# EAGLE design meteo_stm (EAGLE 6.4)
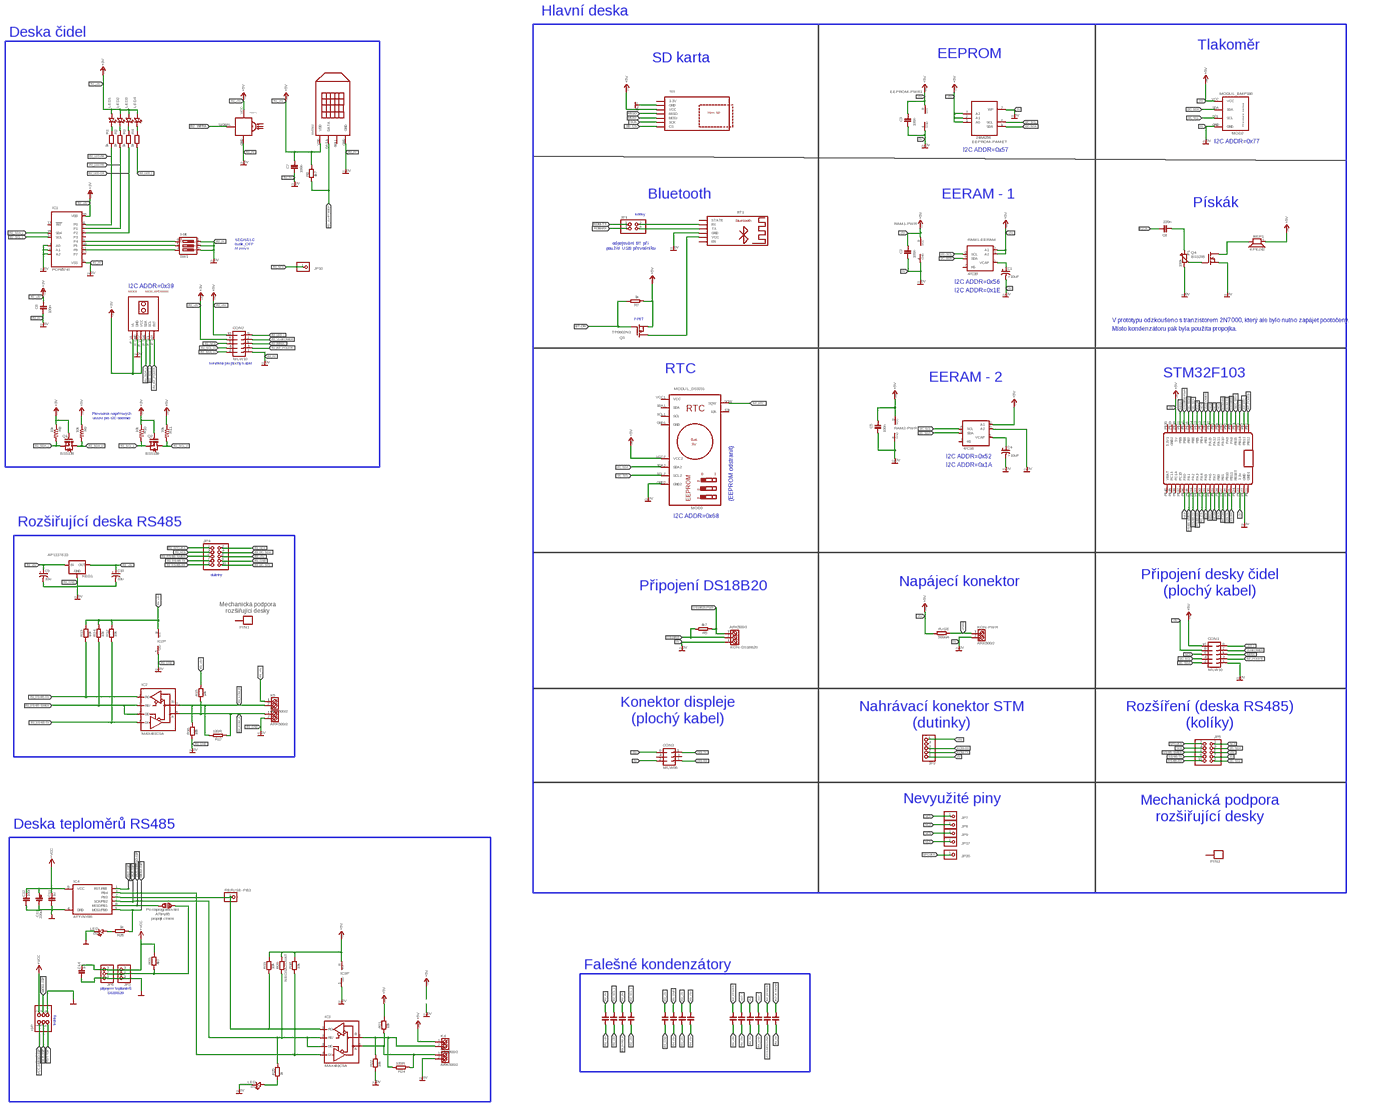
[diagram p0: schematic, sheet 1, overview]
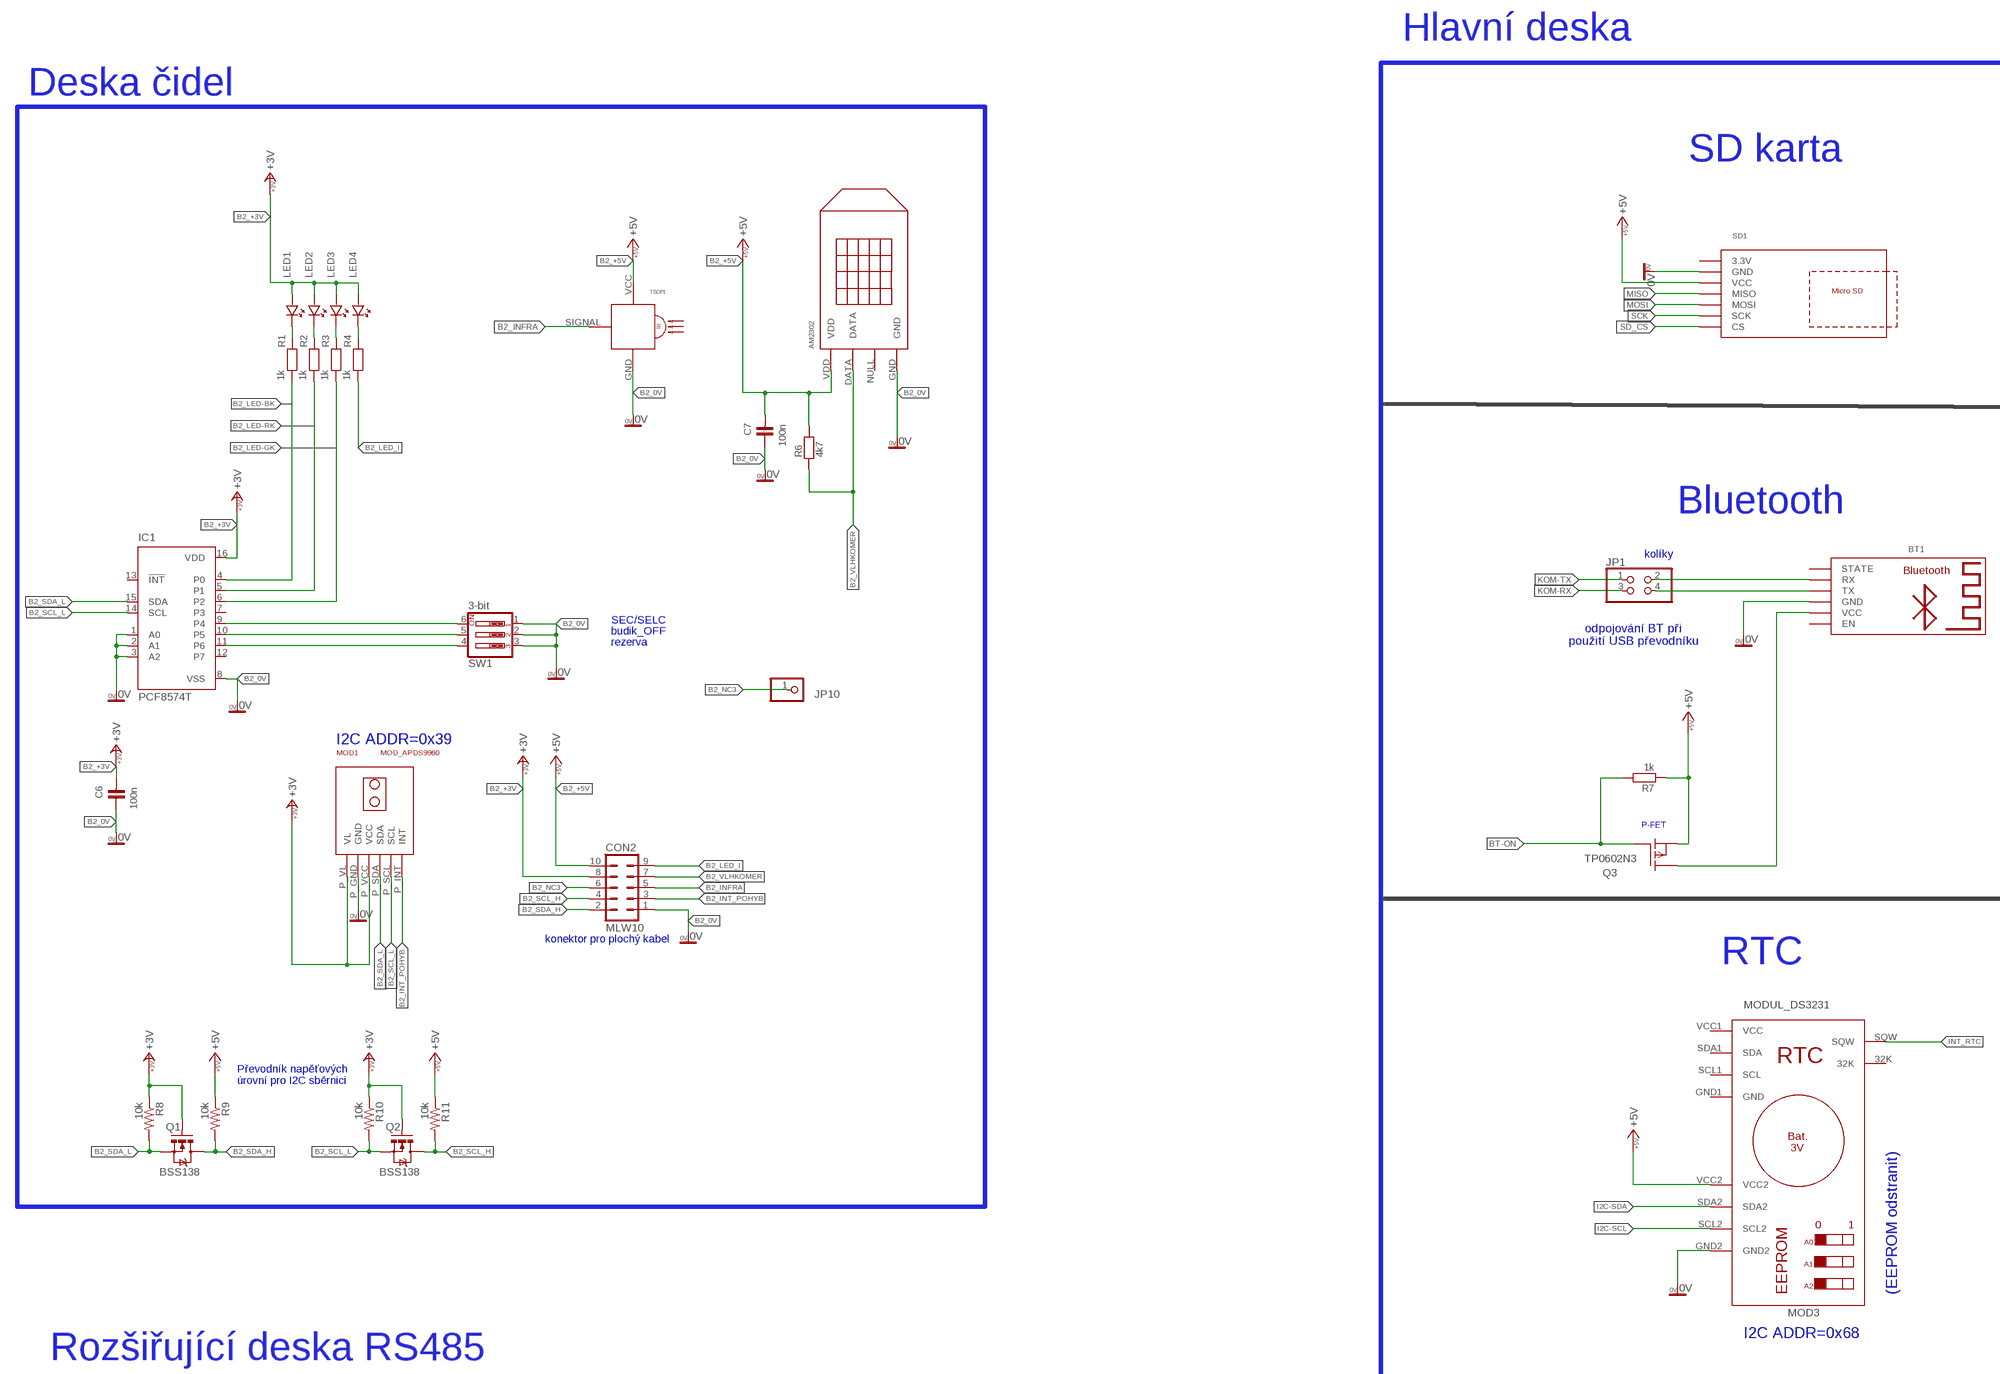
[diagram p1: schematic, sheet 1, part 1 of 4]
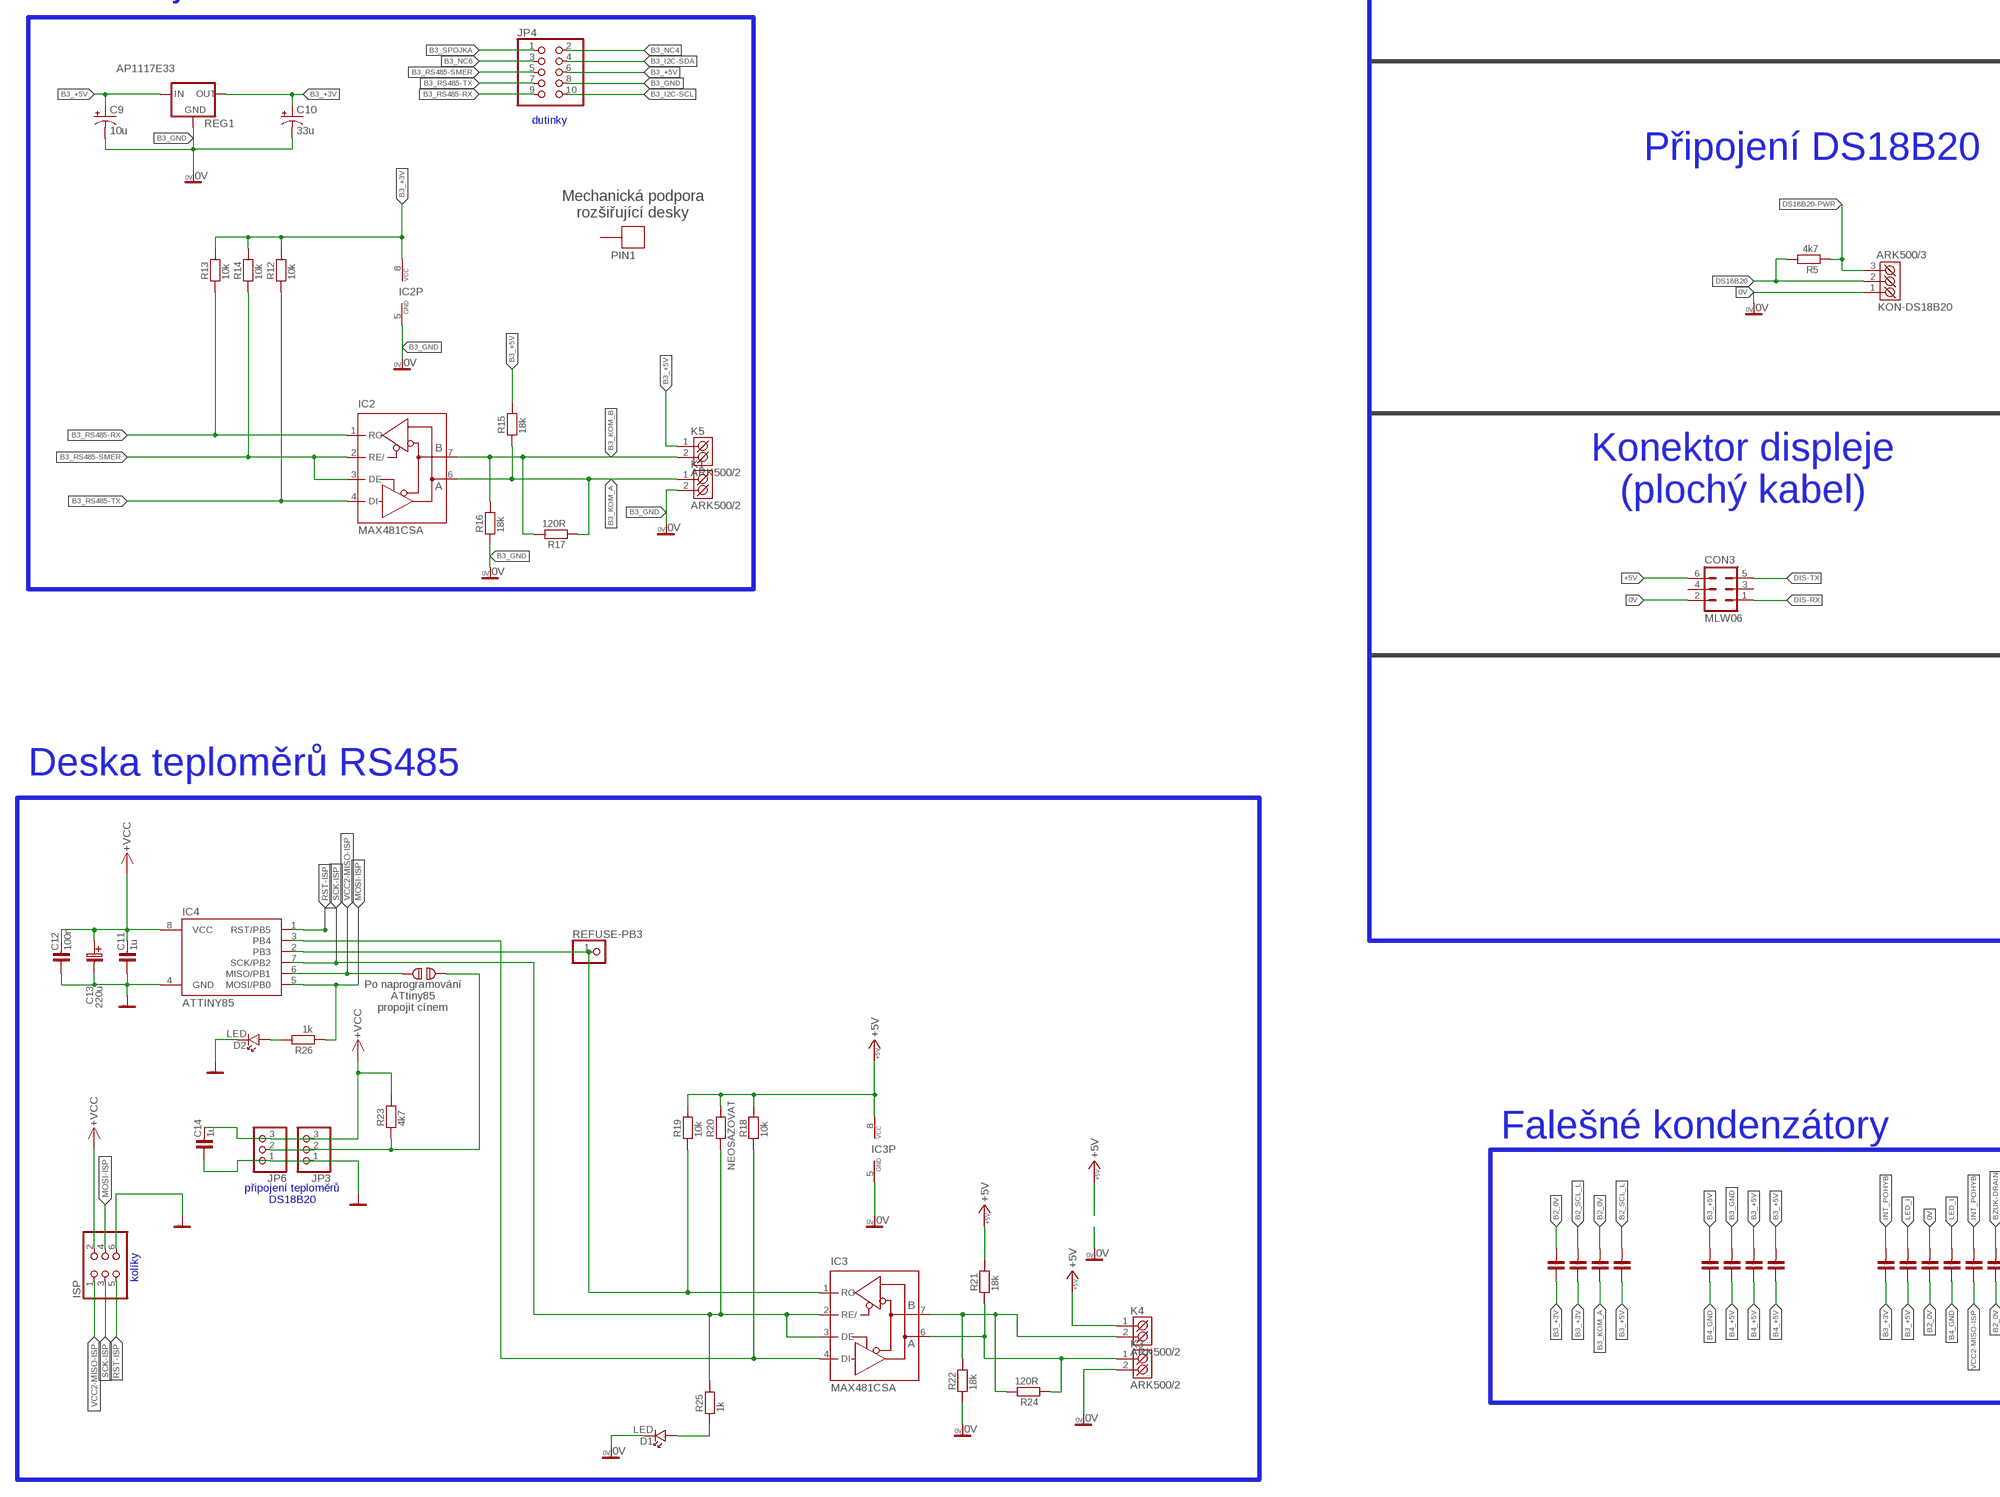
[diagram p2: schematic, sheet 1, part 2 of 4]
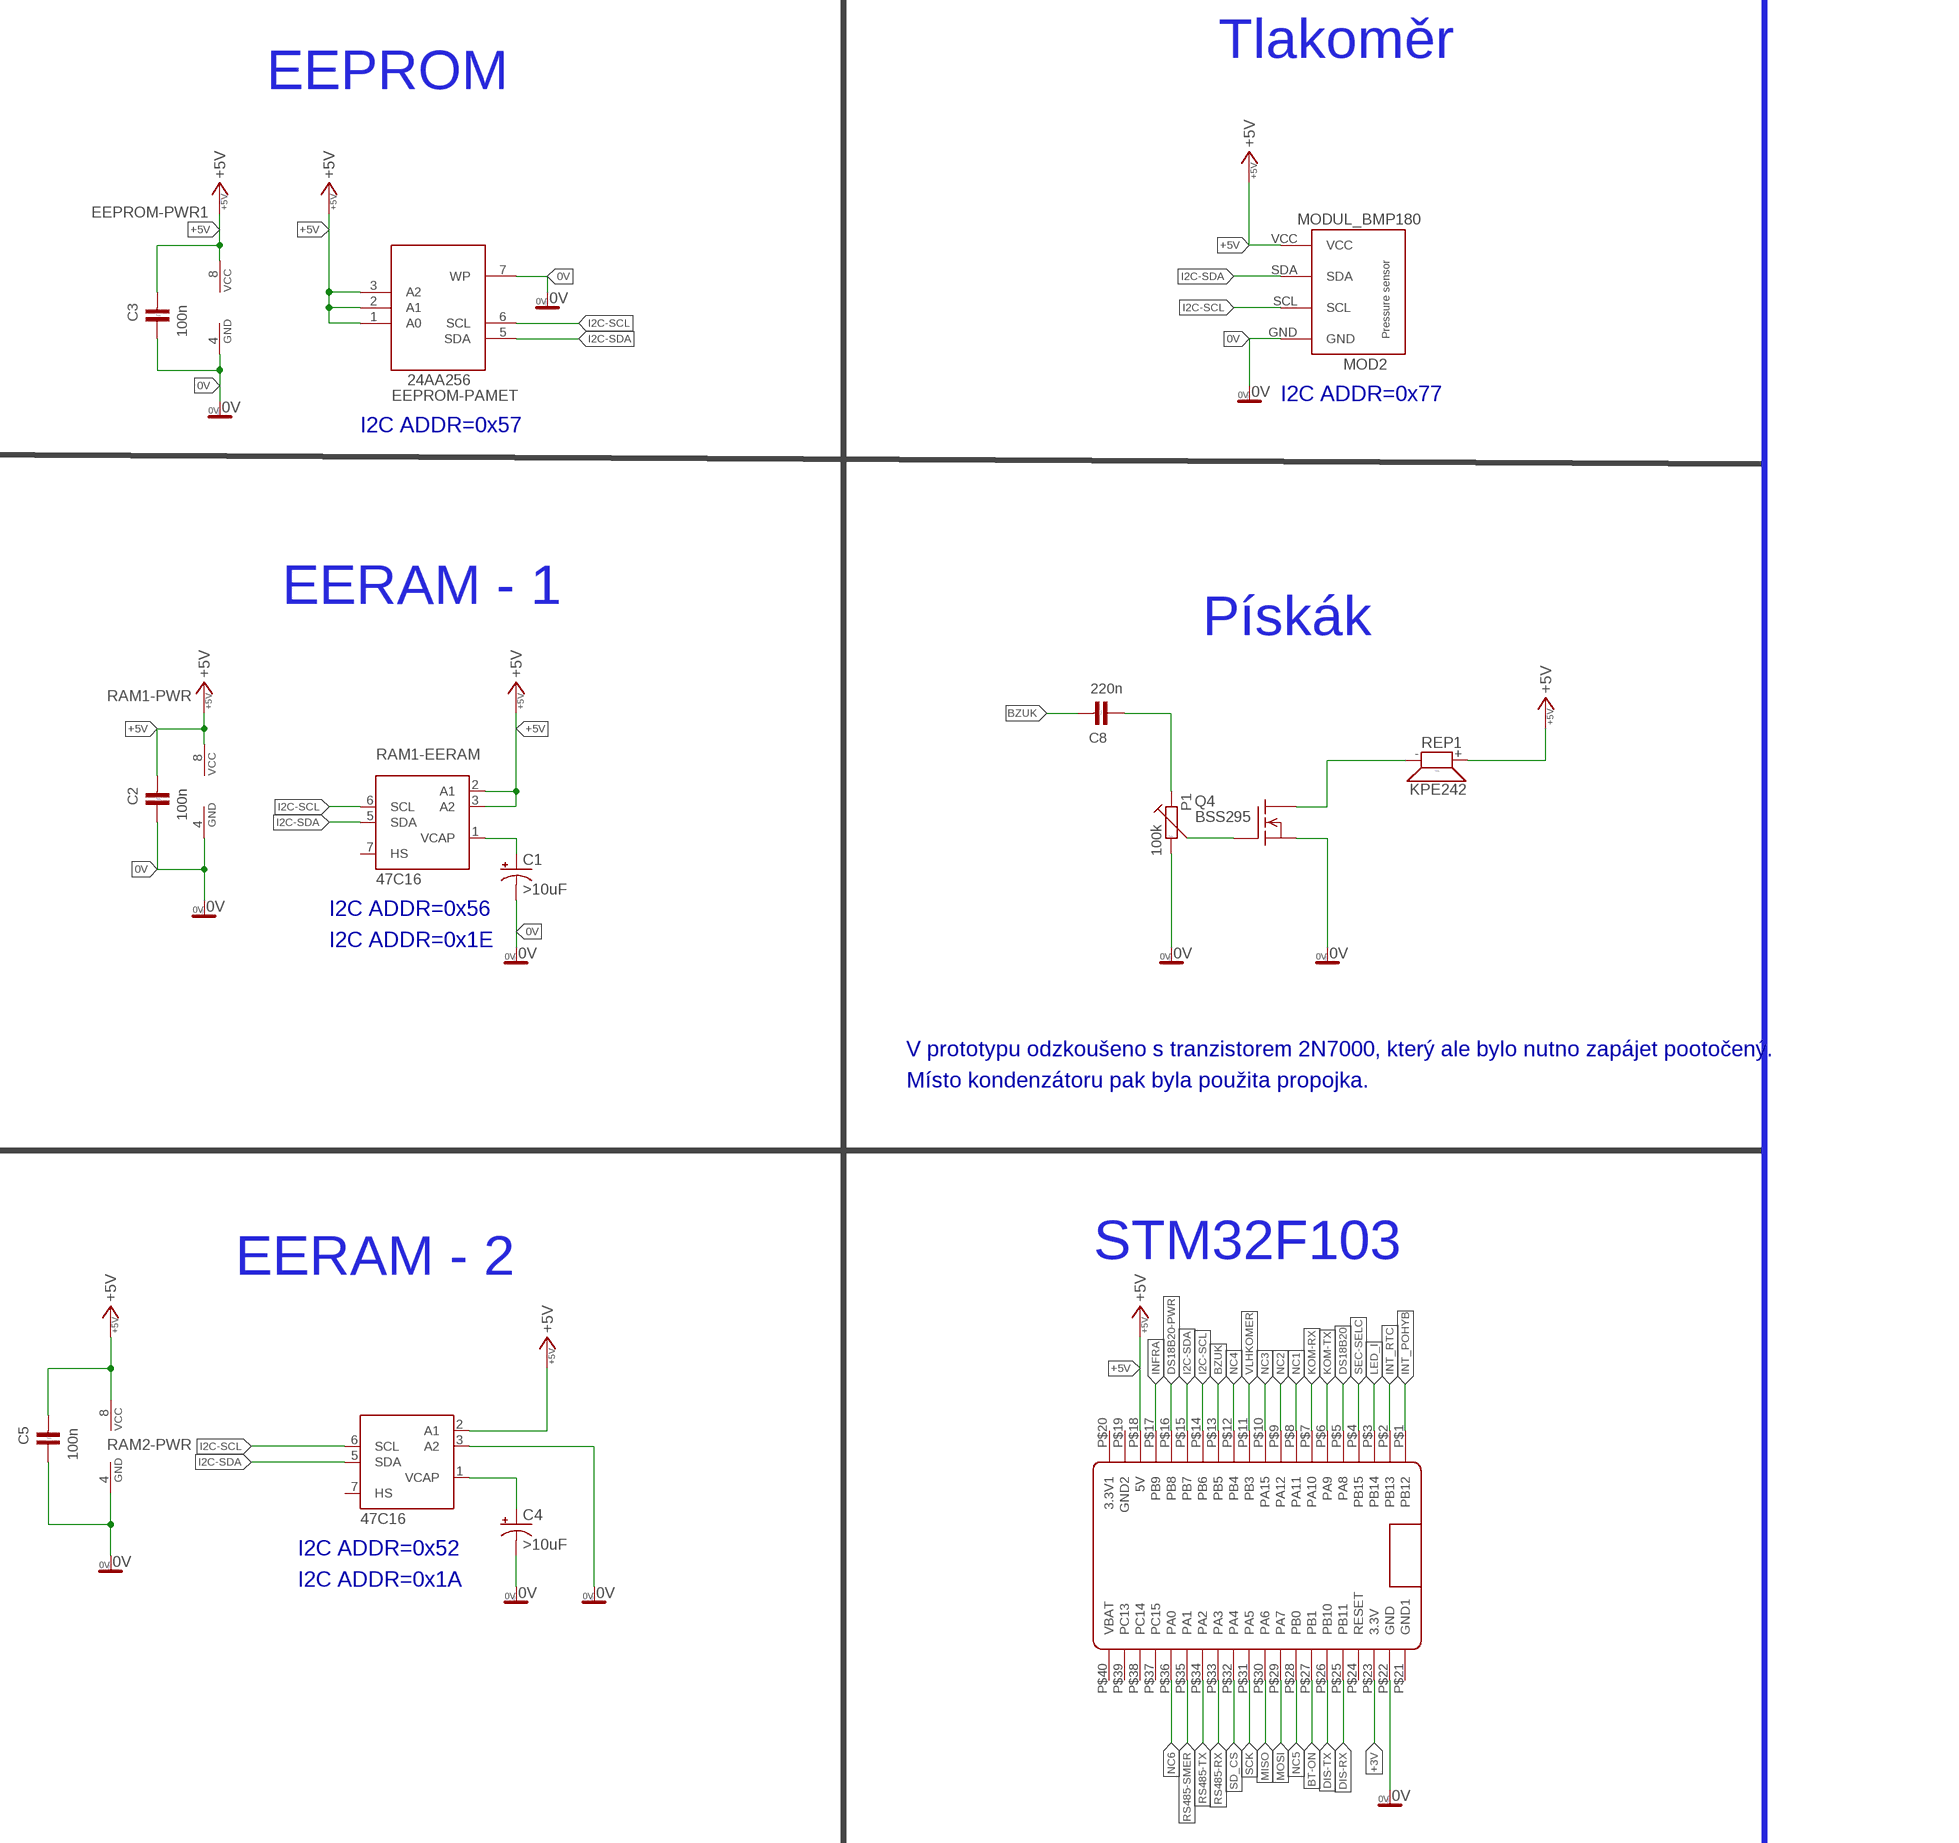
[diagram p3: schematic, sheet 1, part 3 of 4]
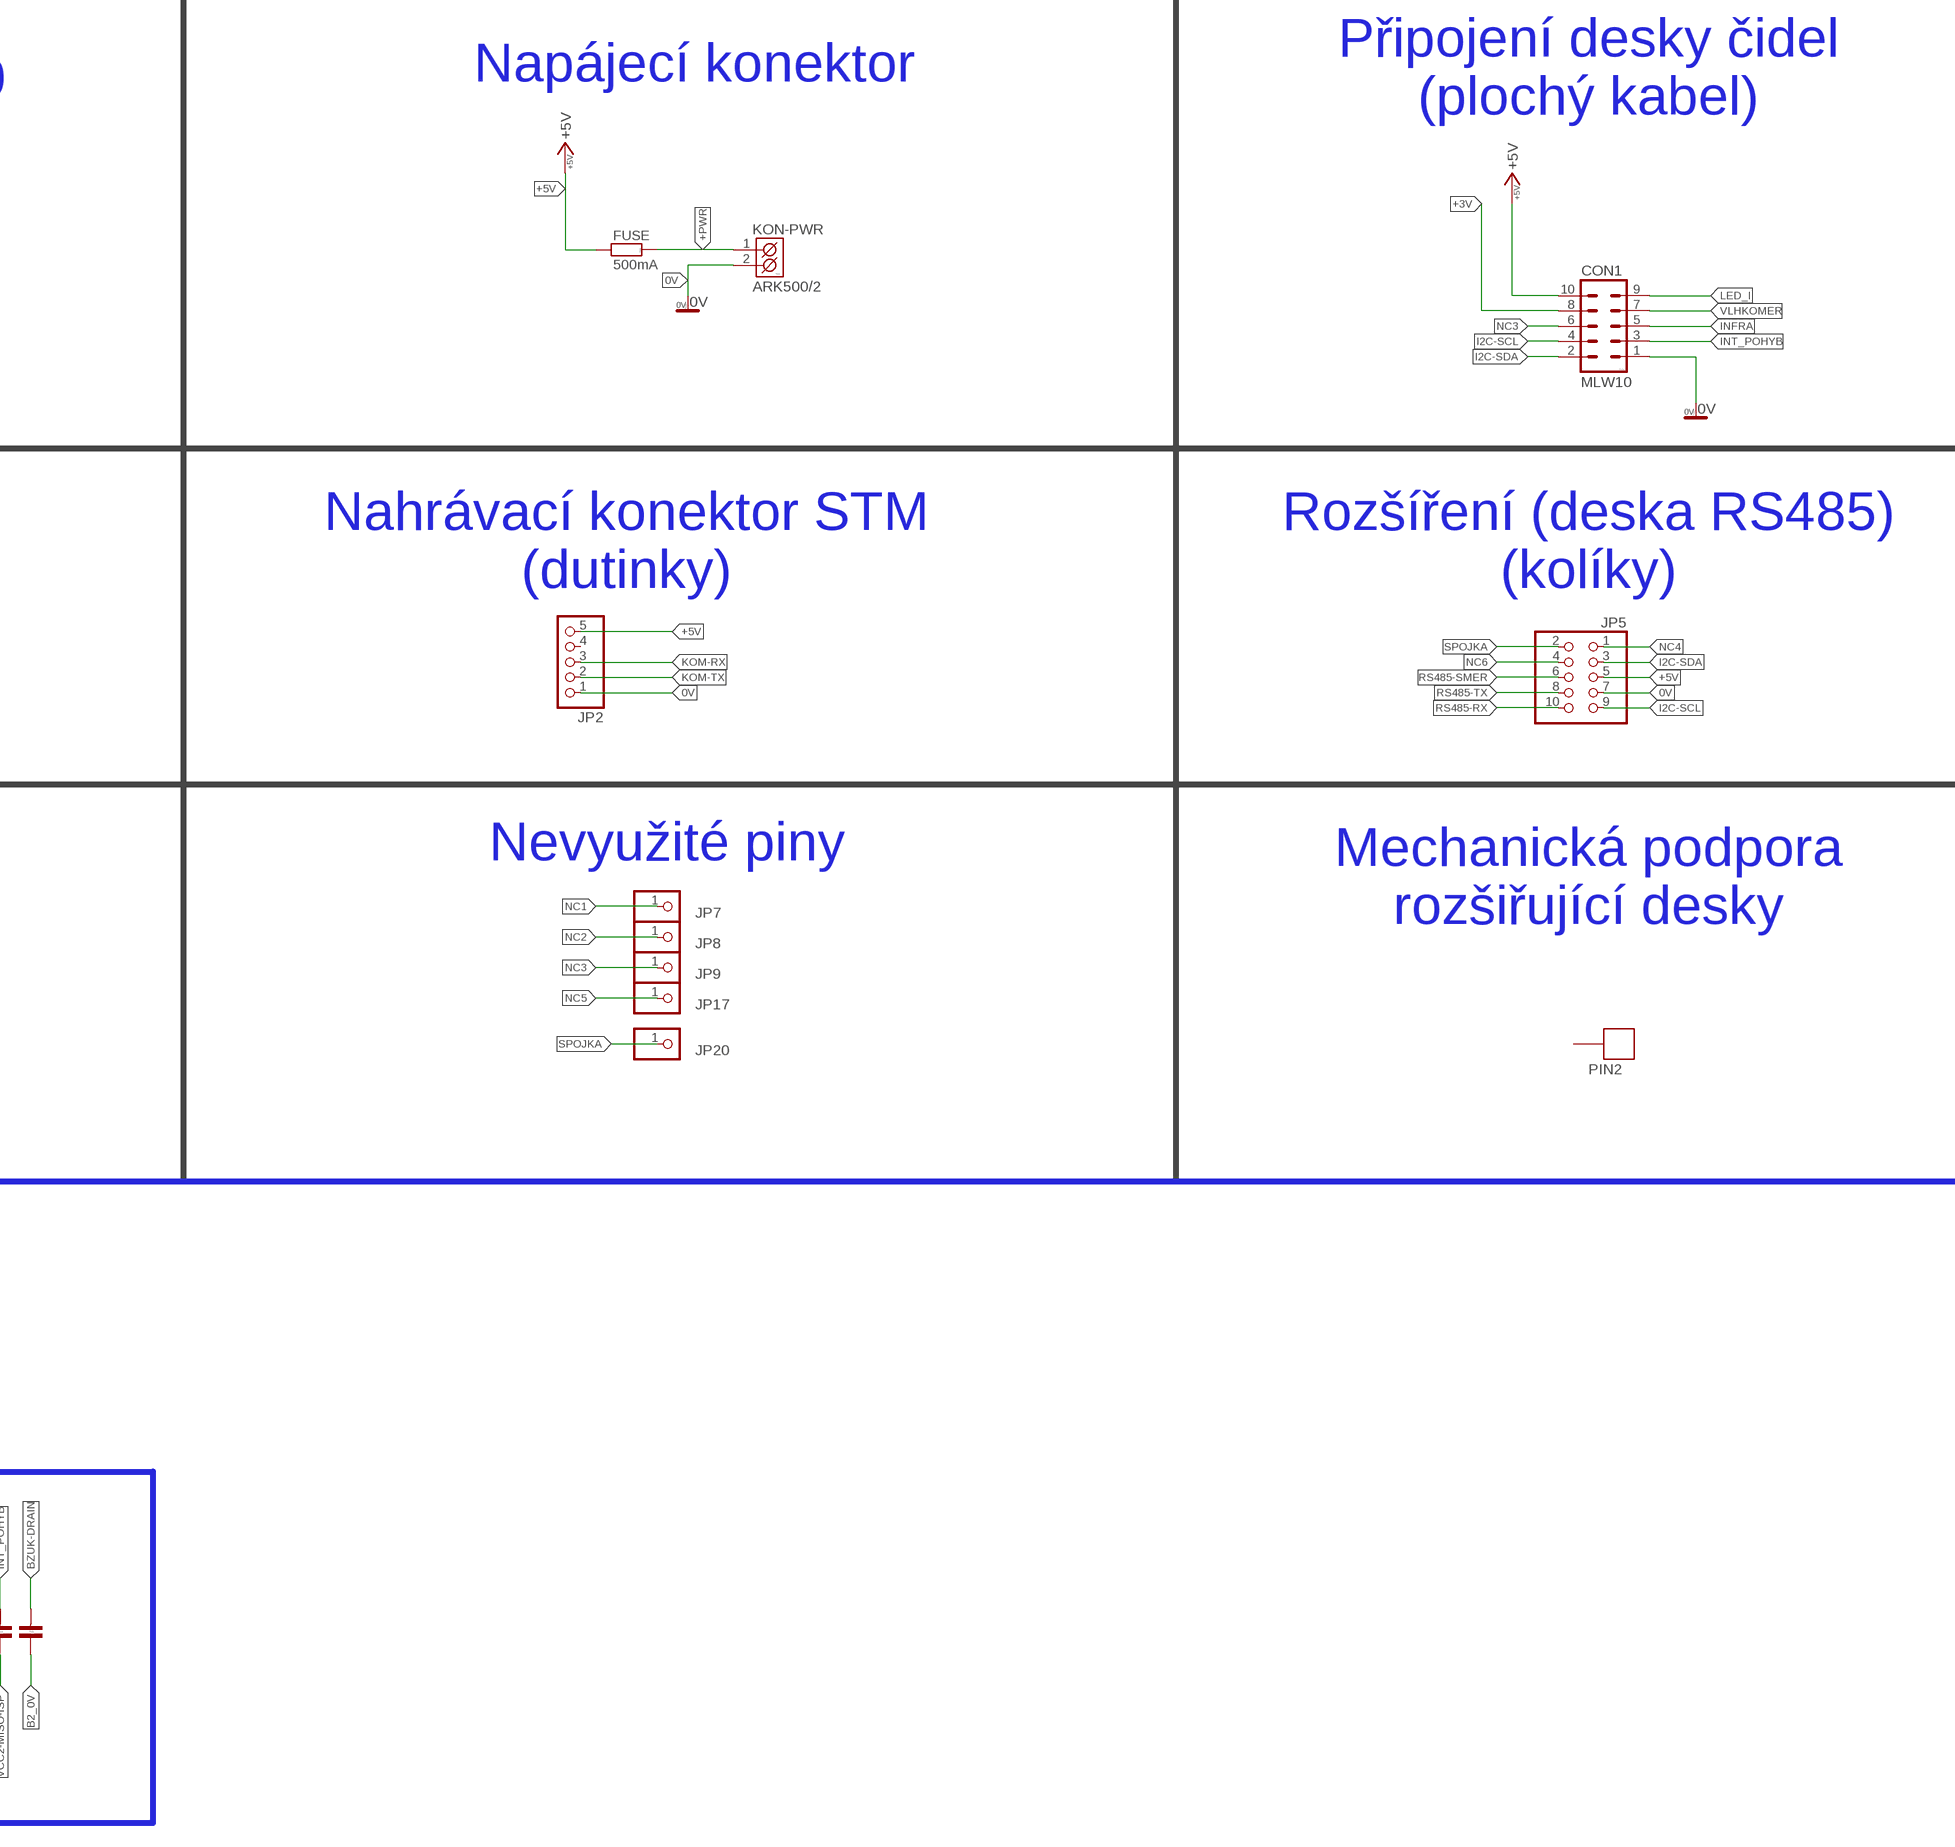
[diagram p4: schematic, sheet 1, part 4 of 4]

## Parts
AM2302  RHT03_DHT-22_AM2302RA  [RHT03_DHT-22/RA]
BT1  BT_MODUL  [BT_MODUL]
C1  >10uF  10UF-POLAR-RADIAL-2.5MM-25V-20%  [CPOL-RADIAL-2.5MM-5MM]
C2  100n  C-KERAMIK_SMD_0805  [0805]
C3  100n  C-KERAMIK_SMD_0805  [0805]
C4  >10uF  10UF-POLAR-RADIAL-2.5MM-25V-20%  [CPOL-RADIAL-2.5MM-5MM]
C5  100n  C-KERAMIK_SMD_0805  [0805]
C6  100n  C-KERAMIK_SMD_0805  [0805]
C7  100n  C-KERAMIK_SMD_0805  [0805]
C8  220n  C-KERAMIK_SMD_0805  [0805]
C9  10u  10UF-POLAR-RADIAL-2.5MM-25V-20%  [CPOL-RADIAL-2.5MM-5MM]
C10  33u  10UF-POLAR-RADIAL-2.5MM-25V-20%  [CPOL-RADIAL-2.5MM-5MM]
C11  1u  C-KERAMIK_SMD_0805  [0805]
C12  100n  C-KERAMIK_SMD_0805  [0805]
C13  220u  C-ELEKTROLYT_3,5  [C-EL_3,5]
C14  1u  C-KERAMIK_SMD_0805  [0805]
C15  ---  C-KERAMIK_SMD_0805  [0805]
C16  ---  C-KERAMIK_SMD_0805  [0805]
C17  ---  C-KERAMIK_SMD_0805  [0805]
C18  ---  C-KERAMIK_SMD_0805  [0805]
C19  ---  C-KERAMIK_SMD_0805  [0805]
C20  ---  C-KERAMIK_SMD_0805  [0805]
C21  ---  C-KERAMIK_SMD_0805  [0805]
C22  ---  C-KERAMIK_SMD_0805  [0805]
C23  ---  C-KERAMIK_SMD_0805  [0805]
C24  ---  C-KERAMIK_SMD_0805  [0805]
C25  ---  C-KERAMIK_SMD_0805  [0805]
C26  ---  C-KERAMIK_SMD_0805  [0805]
C27  ---  C-KERAMIK_SMD_0805  [0805]
C28  ---  C-KERAMIK_SMD_0805  [0805]
CON1  MLW10  [MLW10G]
CON2  MLW10  [MLW10G]
CON3  MLW06  [MLW06G]
D1  LED  LED_SMD_1206  [P1206]
D2  LED  LED_SMD_1206  [P1206]
EEPROM  24AA256  EEPROM  [SO8]
FUSE  500mA  R_SMD_1206  [1206]
IC1  PCF8574T  [SO16W]
IC2  MAX481CSA  [SO08]
IC3  MAX481CSA  [SO08]
IC4  ATTINY85  ATTINY85SU  [ATTINY85]
ISP  PINHD-2X3  [2X03]
JP1  PINHD-2X2  [2X02]
JP2  PINHD-1X5  [1X05]
JP3  PINHD-1X3  [1X03]
JP4  PINHD-2X5  [2X05]
JP5  PINHD-2X5  [2X05]
JP6  PINHD-1X3  [1X03]
JP7  PINHD-1X1  [1X01]
JP8  PINHD-1X1  [1X01]
JP9  PINHD-1X1  [1X01]
JP10  PINHD-1X1  [1X01]
JP17  PINHD-1X1  [1X01]
JP20  PINHD-1X1  [1X01]
K1  ARK500/2  [ARK500/2]
K3  ARK500/2  [ARK500/2]
K4  ARK500/2  [ARK500/2]
K5  ARK500/2  [ARK500/2]
KON-DS18B20  ARK500/3  [ARK500/3]
KON-PWR  ARK500/2  [ARK500/2]
LED1  Modra  LED_3  [LED_3]
LED2  Cervena  LED_3  [LED_3]
LED3  Zelena  LED_3  [LED_3]
LED4  Bila  LED_3  [LED_3]
MOD1  MOD_APDS9960  [MOD_APDS9960]
MOD2  MODUL_BMP180  [MODUL_BMP180]
MOD3  MODUL_DS3231  [DS3231]
P1  100k  TRIMR64Y  [64Y]
PIN1  BIGPIN  [BIGPIN]
PIN2  BIGPIN  [BIGPIN]
Q1  BSS138  MOSFET-NCHANNELSMD  [SOT23-3]
Q2  BSS138  MOSFET-NCHANNELSMD  [SOT23-3]
Q3  TP0602N3  [TO-92]
Q4  BSS295  [TO92]
R1  1k  R_SMD_0805  [0805]
R2  1k  R_SMD_0805  [0805]
R3  1k  R_SMD_0805  [0805]
R4  1k  R_SMD_0805  [0805]
R5  4k7  R_SMD_0805  [0805]
R6  4k7  R_SMD_0805  [0805]
R7  1k  R_SMD_0805  [0805]
R8  10k  RESISTOR0805-RES  [0805]
R9  10k  RESISTOR0805-RES  [0805]
R10  10k  RESISTOR0805-RES  [0805]
R11  10k  RESISTOR0805-RES  [0805]
R12  10k  R_SMD_0805  [0805]
R13  10k  R_SMD_0805  [0805]
R14  10k  R_SMD_0805  [0805]
R15  18k  R_SMD_0805  [0805]
R16  18k  R_SMD_0805  [0805]
R17  120R  R_SMD_0805  [0805]
R18  10k  R_SMD_0805  [0805]
R19  10k  R_SMD_0805  [0805]
R20  NEOSAZOVAT  R_SMD_0805  [0805]
R21  18k  R_SMD_0805  [0805]
R22  18k  R_SMD_0805  [0805]
R23  4k7  R_SMD_0805  [0805]
R24  120R  R_SMD_0805  [0805]
R25  1k  R_SMD_0805  [0805]
R26  1k  R_SMD_0805  [0805]
RAM1  47C16  PCA8581CT  [SO08]
RAM2  47C16  PCA8581CT  [SO08]
REFUSE-PB3  PINHD-1X1  [1X01]
REG1  AP1117E33  V_REG_LD1117VXXLD1117-SMD  [SOT223]
REP1  KPE242  [KPE242]
SD1  MICROSD_MODUL  [MICROSD_MODUL]
SJ-SCL1  SJ  SOLDERJUMPER  [SJ_2S-NO]
SW1  3-bit  SW_DIP-3  [EDG-03]
TSOP1  TSOP  [TSOP]
U$1  BLUE_PILL  [BLUE_PILL]

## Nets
0V: BT1.GND C1.2(-) C2.1 C3.1 C4.2(-) C5.1 C24.2 CON1.1 CON3.2 EEPROM.4(-PWR1:GND) EEPROM.7(-PAMET:WP) JP2.1 JP5.7 KON-DS18B20.1(K1) KON-PWR.2(K2) MOD2.GND MOD3.GND2 P1.2 Q4.3(S) RAM1.4(-PWR:GND) RAM2.3(-EERAM:A2) RAM2.4(-PWR:GND) SD1.GND U$1.P$22(GND)
+3V: CON1.8 U$1.P$23(3.3V)
+5V: C2.2 C3.2 C5.2 CON1.10 CON3.6 EEPROM.1(-PAMET:A0) EEPROM.2(-PAMET:A1) EEPROM.3(-PAMET:A2) EEPROM.8(-PWR1:VCC) FUSE.1 JP2.5 JP5.5 MOD2.VCC MOD3.VCC2 Q3.1(S) R7.1 RAM1.2(-EERAM:A1) RAM1.3(-EERAM:A2) RAM1.8(-PWR:VCC) RAM2.2(-EERAM:A1) RAM2.8(-PWR:VCC) REP1.+ SD1.VCC U$1.P$18(5V)
+PWR: FUSE.2 KON-PWR.1(K1)
B2_0V: AM2302.GND C6.1 C7.1 C15.2 C22.2 C24.1 C28.1 CON2.1 IC1.1(A0) IC1.2(A1) IC1.3(A2) IC1.8(VSS) MOD1.P_GND(GND) SW1.1 SW1.2 SW1.3 TSOP1.GND ; supply symbol labelled 0V
B2_+3V: C6.2 CON2.8 IC1.16(VDD) LED1.A LED2.A LED3.A LED4.A MOD1.P_VCC(VCC) MOD1.P_VL(VL) Q1.1(G) Q2.1(G) R8.1 R10.1 ; supply symbol labelled +3V
B2_+5V: AM2302.VDD C7.2 CON2.10 R6.2 R9.1 R11.1 TSOP1.VCC ; supply symbol labelled +5V
B2_INFRA: CON2.5 TSOP1.SIGNAL
B2_INT_POHYB: CON2.3 MOD1.P_INT(INT)
B2_LED-BK: IC1.4(P0) R1.1
B2_LED-GK: IC1.6(P2) R3.1
B2_LED-RK: IC1.5(P1) R2.1
B2_LED_I: CON2.9 R4.1
B2_NC3: CON2.6 JP10.1
B2_SCL_H: CON2.4 Q2.3(D) R11.2
B2_SCL_L: C16.2 C18.2 IC1.14(SCL) MOD1.P_SCL(SCL) Q2.2(S) R10.2
B2_SDA_H: CON2.2 Q1.3(D) R9.2
B2_SDA_L: IC1.15(SDA) MOD1.P_SDA(SDA) Q1.2(S) R8.2
B2_VLHKOMER: AM2302.DATA CON2.7 R6.1
B3_+3V: C10.1(+) C18.1 C21.1 C22.1 IC2.8(VCC) R12.2 R13.2 R14.2 REG1.2(OUT)
B3_+5V: C9.1(+) C16.1 C17.2 C20.2 C23.2 C25.1 JP4.6 K5.1(K1) R15.2 REG1.3(IN)
B3_GND: C9.2(-) C10.2(-) C19.2 IC2.5(GND) JP4.8 K1.2(K2) R16.1 REG1.1(GND) ; supply symbol labelled 0V
B3_I2C-SCL: JP4.10
B3_I2C-SDA: JP4.4
B3_KOM_A: C15.1 IC2.6(A) K1.1(K1) R15.1 R17.1
B3_KOM_B: IC2.7(B) K5.2(K2) R16.2 R17.2
B3_NC4: JP4.2
B3_NC6: JP4.3
B3_RS485-RX: IC2.1(RO) JP4.9 R13.1
B3_RS485-SMER: IC2.2(RE/) IC2.3(DE) JP4.5 R14.1
B3_RS485-TX: IC2.4(DI) JP4.7 R12.1
B3_SPOJKA: JP4.1
B4_+5V: C11.2 C12.2 C13.C+(C_EL+) C14.2 C19.1 C20.1 C23.1 IC3.8(VCC) IC4.8(VCC) ISP.2 JP3.3 JP6.3 K4.1(K1) R18.2 R19.2 R20.2 R21.2 R23.2 ; supply symbol labelled +5V, +VCC
B4_A: IC3.6(A) K3.1(K1) R21.1 R24.1
B4_B: IC3.7(B) K4.2(K2) R22.2 R24.2
B4_GND: C11.1 C12.1 C13.C-(C_EL-) C14.1 C17.1 C26.1 D1.K D2.K IC3.5(GND) IC4.4(GND) ISP.6 JP3.1 JP6.1 K3.2(K2) R22.1 ; supply symbol labelled GND, 0V
BLUE-RX: BT1.RX JP1.2
BLUE-TX: BT1.TX JP1.4
BT-ON: Q3.2(G) R7.2 U$1.P$27(PB1)
BT-PWR: BT1.VCC Q3.3(D)
BZUK: C8.2 U$1.P$13(PB5)
BZUK-C: C8.1 P1.1
BZUK-DRAIN: C28.2 Q4.2(D) REP1.-
BZUK-GATE: P1.3 Q4.1(G)
DIS-RX: CON3.1 U$1.P$25(PB11)
DIS-TX: CON3.5 U$1.P$26(PB10)
DS18B20: KON-DS18B20.2(K2) R5.2 U$1.P$5(PA8)
DS18B20-PWR: KON-DS18B20.3(K3) R5.1 U$1.P$16(PB8)
I2C-SCL: CON1.4 EEPROM.6(-PAMET:SCL) JP5.9 MOD2.SCL MOD3.SCL2 RAM1.6(-EERAM:SCL) RAM2.6(-EERAM:SCL) U$1.P$14(PB6)
I2C-SDA: CON1.2 EEPROM.5(-PAMET:SDA) JP5.3 MOD2.SDA MOD3.SDA2 RAM1.5(-EERAM:SDA) RAM2.5(-EERAM:SDA) U$1.P$15(PB7)
INFRA: CON1.5 U$1.P$17(PB9)
INT_POHYB: C21.2 C27.2 CON1.3 U$1.P$1(PB12)
INT_RTC: MOD3.SQW U$1.P$2(PB13)
KOM-RX: JP1.3 JP2.3 U$1.P$7(PA10)
KOM-TX: JP1.1 JP2.2 U$1.P$6(PA9)
LED_I: C25.2 C26.2 CON1.9 U$1.P$3(PB14)
MISO: SD1.MISO U$1.P$30(PA6)
MOSI: SD1.MOSI U$1.P$29(PA7)
MOSI-ISP: IC4.5(MOSI/PB0) ISP.4 R26.1
N$1: LED1.K R1.2
N$2: LED2.K R2.2
N$3: LED3.K R3.2
N$5: LED4.K R4.2
N$6: D2.A R26.2
N$7: IC1.11(P6) SW1.4
N$8: C4.1(+) RAM2.1(-EERAM:VCAP)
N$9: IC1.10(P5) SW1.5
N$10: IC1.9(P4) SW1.6
N$12: JP3.2 JP6.2 R23.1 SJ-SCL1.2
N$13: D1.A R25.1
N$17: C1.1(+) RAM1.1(-EERAM:VCAP)
NC1: JP7.1 U$1.P$8(PA11)
NC2: JP8.1 U$1.P$9(PA12)
NC3: CON1.6 JP9.1 U$1.P$10(PA15)
NC4: JP5.1 U$1.P$12(PB4)
NC5: JP17.1 U$1.P$28(PB0)
NC6: JP5.4 U$1.P$36(PA0)
RS485-RX: JP5.10 U$1.P$33(PA3)
RS485-SMER: JP5.6 U$1.P$35(PA1)
RS485-TX: JP5.8 U$1.P$34(PA2)
RST-ISP: IC4.1(RST/PB5) ISP.5
SCK: SD1.SCK U$1.P$31(PA5)
SCK-ISP: IC3.2(RE/) IC3.3(DE) IC4.7(SCK/PB2) ISP.3 R20.1 R25.2
SD_CS: SD1.CS U$1.P$32(PA4)
SEC-SELC: U$1.P$4(PB15)
SPOJKA: JP5.2 JP20.1
TINY-PB4: IC3.4(DI) IC4.3(PB4) R18.1
TL1: IC3.1(RO) IC4.2(PB3) R19.1 REFUSE-PB3.1
VCC2-MISO-ISP: C27.1 IC4.6(MISO/PB1) ISP.1 SJ-SCL1.1
VLHKOMER: CON1.7 U$1.P$11(PB3)
Unconnected: AM2302.NULL BT1.EN BT1.STATE CON3.3 CON3.4 IC1.7(P3) IC1.12(P7) IC1.13(!INT) JP2.4 MOD3.32K MOD3.GND1(GND) MOD3.SCL1(SCL) MOD3.SDA1(SDA) MOD3.VCC1(VCC) PIN1.P$1 PIN2.P$1 RAM1.7(-EERAM:HS) RAM2.7(-EERAM:HS) U$1.P$19(GND2) U$1.P$20(3.3V1) U$1.P$24(RESET) U$1.P$37(PC15) U$1.P$38(PC14) U$1.P$39(PC13) U$1.P$40(VBAT)

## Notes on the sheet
- Hlavní deska
- Deska čidel
- Tlakoměr
- SD karta | EEPROM
- I2C ADDR=0x77
- I2C ADDR=0x57
- Bluetooth | EERAM - 1
- Pískák
- kolíky
- SEC/SELC
- budik_OFF
- odpojování BT při
  použití USB převodníku
- rezerva
- I2C ADDR=0x56
- I2C ADDR=0x39
- I2C ADDR=0x1E
- P-FET
- V prototypu odzkoušeno s tranzistorem 2N7000, který ale bylo nutno zapájet pootočený.
- Místo kondenzátoru pak byla použita propojka.
- konektor pro plochý kabel
- RTC | STM32F103
- EERAM - 2
- Převodník napěťových
  úrovní pro I2C sběrnici
- I2C ADDR=0x52
- I2C ADDR=0x1A
- (EEPROM odstranit)
- I2C ADDR=0x68
- Rozšiřující deska RS485
- dutinky
- Připojení desky čidel
  (plochý kabel)
- Připojení DS18B20 | Napájecí konektor
- Mechanická podpora
  rozšiřující desky
- Konektor displeje
  (plochý kabel)
- Nahrávací konektor STM
  (dutinky)
- Rozšíření (deska RS485)
  (kolíky)
- Nevyužité piny
- Mechanická podpora
  rozšiřující desky
- Deska teploměrů RS485
- Po naprogramování
  ATtiny85
  propojit cínem
- Falešné kondenzátory
- připojení teploměrů
  DS18B20
- kolíky

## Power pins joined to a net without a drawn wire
3.3V: SD1.3,3(3.3V)
GND1: U$1.P$21(GND1)

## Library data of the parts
AM2302 = RHT03_DHT-22_AM2302:RHT03_DHT-22_AM2302: RHT03 / DHT-22 / AM2302 Packages and symbol for the RHT03 / DHT-22 relative humidity and temperature sensor. Note: The AM2302 is a wired version of the DHT-22 which typically requires less clearance and is thus provided as a separate package.; PROD_ID: SEN-10167
BT1 = BT_modul:BT_MODUL: BT modul
C1 C4 C9 C10 = SparkFun-Capacitors:10UF-POLAR: 10.0µF polarized capacitors; PROD_ID: CAP-08440; VALUE: 10uF
C2 C3 C5-C8 C11 C12 C14-C28 = #PaJa_30:C-KERAMIK: Kondenzator - keramicky
C13 = #PaJa_30:C-ELEKTROLYT: Kondenzator - elektrolyticky
CON1 CON2 = #PaJa_konektory:MLW10: Konektory MLW - vidlice - 10x
CON3 = #PaJa_konektory:MLW06: Konektory MLW - vidlice - 6x
D1 D2 LED1-LED4 = #PaJa_30:LED: LED - jednobarevna
EEPROM = eeprom:EEPROM: EEPROM
FUSE R1-R7 R12-R26 = #PaJa_30:R: Rezistor
IC1 = micro-philips:PCF8574: I2C-Bus Remote 8-bit I/O expander http://www.semiconductors.philips.com/acrobat_download/datasheets/PCF8574_4.pdf
IC2 IC3 = maxim:MAX481CSA: RS485 TRANSEIVER; MF: MAXIM; MPN: MAX481CSA; OC_FARNELL: unknown; OC_NEWARK: 90C3817
IC4 = attiny85:ATTINY85: ATMEL ATtiny 85
ISP = pinhead:PINHD-2X3: PIN HEADER
JP1 = pinhead:PINHD-2X2: PIN HEADER
JP2 = pinhead:PINHD-1X5: PIN HEADER
JP3 JP6 = pinhead:PINHD-1X3: PIN HEADER
JP4 JP5 = pinhead:PINHD-2X5: PIN HEADER
JP7-JP10 JP17 JP20 REFUSE-PB3 = pinhead:PINHD-1X1: PIN HEADER
K1 K3-K5 KON-PWR = #PaJa_konektory:ARK500/2: Svorkovnice - roztec 5mm - dvojita
KON-DS18B20 = #PaJa_konektory:ARK500/3: Svorkovnice - roztec 5mm - trojita
MOD1 = mod_APDS9960:MOD_APDS9960: modul APDS9960
MOD2 = modul_bmp180:MODUL_BMP180
MOD3 = modul_DS3231:MODUL_DS3231: Modul DS3231 s externi pameti
P1 = #PaJa_30:TRIMR: Trimr
PIN1 PIN2 = bigpin:BIGPIN: Jeden ovalny pin
Q1 Q2 = SparkFun:MOSFET-NCHANNEL
Q3 = transistor-fet:TP0602N3: P-Channel Enhancement MOSFET -20V; -2A; 2,0Ohm
Q4 = transistor-fet:BSS295: N-Channel Enhancement MOSFET not checked
R8-R11 = SparkFun:RESISTOR: Resistor
RAM1 RAM2 = i2c:PCA8581: 2048 x 8-Bit EERAM with I²C Bus Interface
REG1 = SparkFun-IC-Power:V_REG_LD1117VXX: LD1117VXX voltage regulator. We carry the 3.3V version (COM-00526) in TO-220 package.; PROD_ID: VREG-13917
REP1 = #PaJa_30:KPE242: Piezo-sirenka - 70dB - 3V az 16V
SD1 = microSD_modul:MICROSD_MODUL: Modul micro SD karty
SJ-SCL1 = solderjump:SOLDERJUMPER: Pájecí propojka
SW1 = special:SW_DIP-3: DIP SWITCH
TSOP1 = TSOP-infra:TSOP: Infra čidlo TSOP...
U$1 = BluePill:BLUE_PILL

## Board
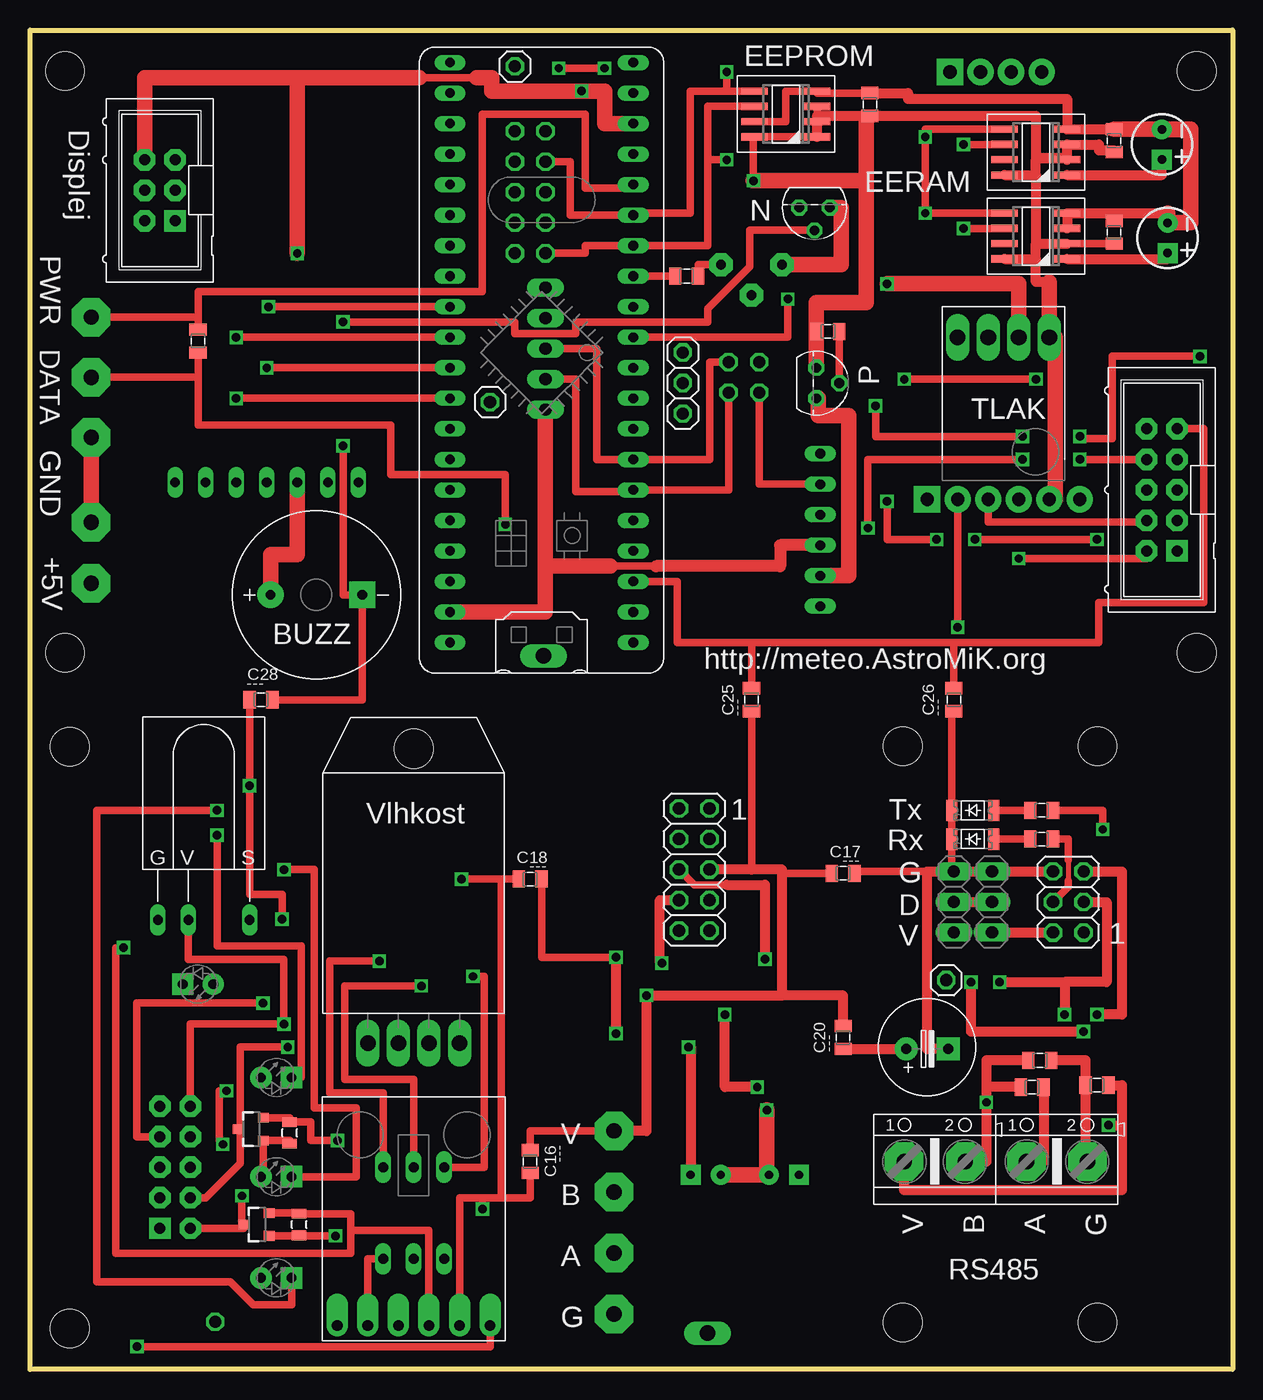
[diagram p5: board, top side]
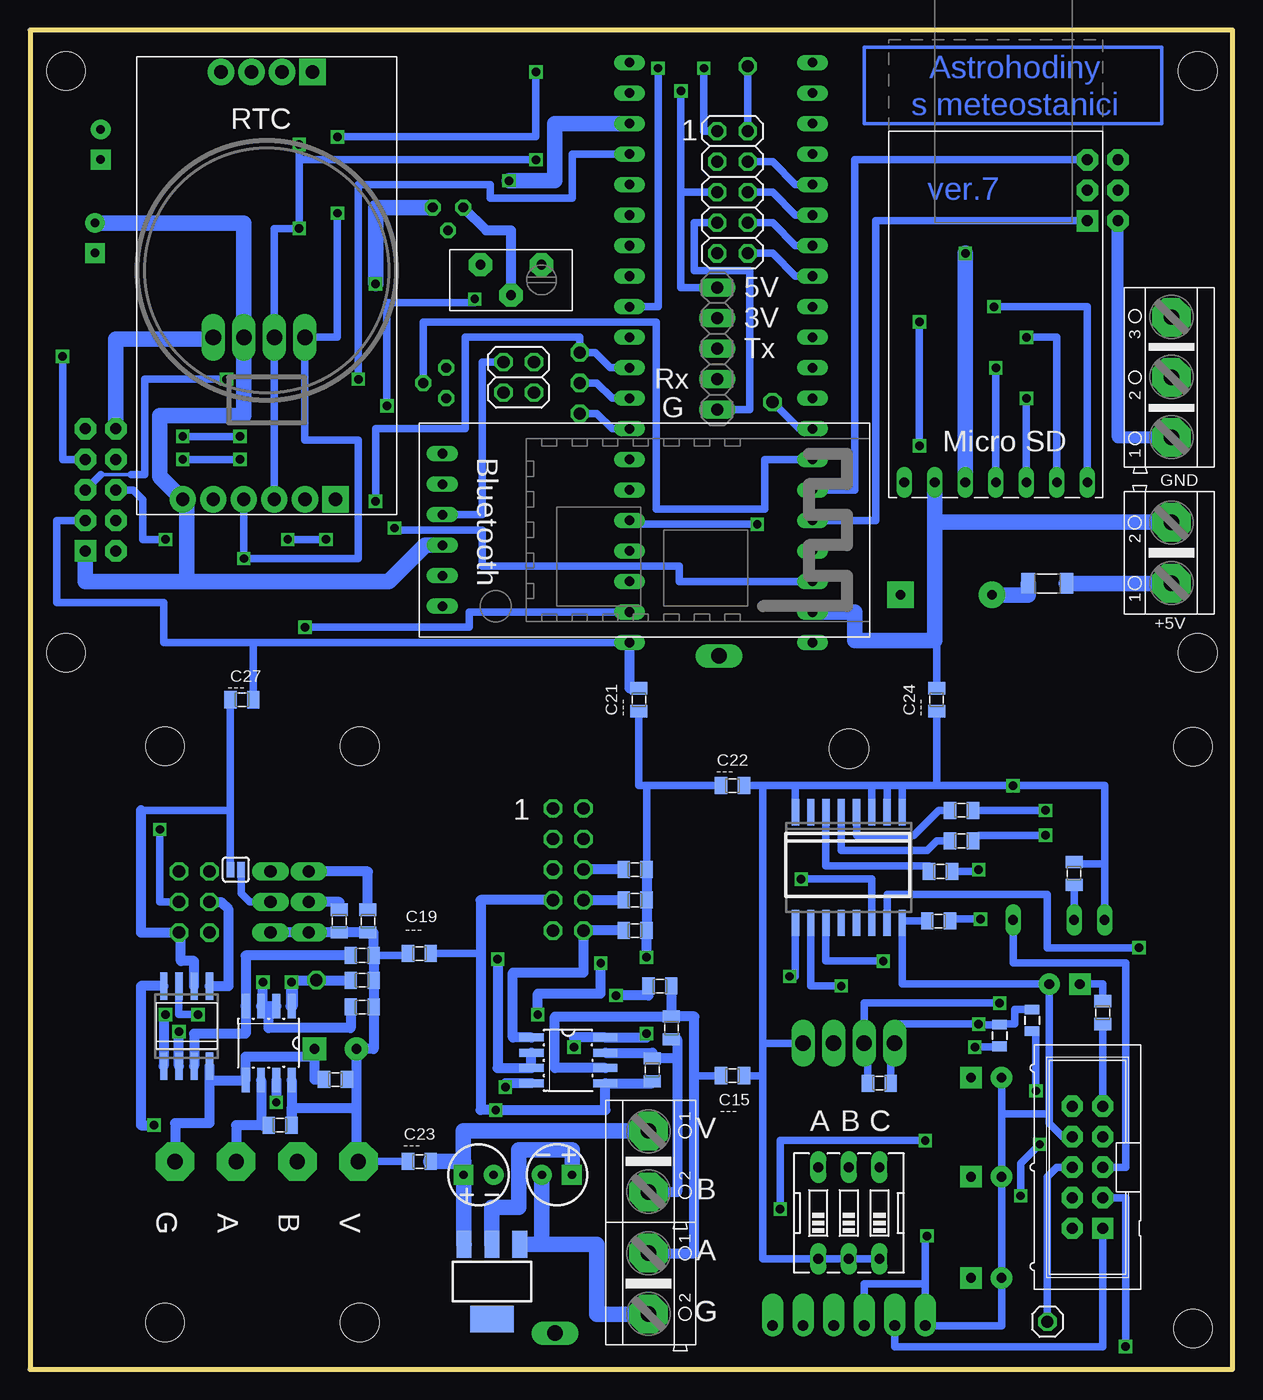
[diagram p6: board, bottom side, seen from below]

Size 100.01 x 111.44 mm. Coordinates in mm from the lower left corner, seen from the top.
Outline: 0,111.44 100.01,111.44 100.01,0 0,0 0,111.44
Copper layers (1*16): Top 0.035mm / dielectric 1.5mm / Bottom 0.035mm
Design rules "default *": minimum track width 10mil, minimum drill 24mil, track to track 8mil, track to pad 8mil, pad to pad 8mil, via to via 8mil, smd to smd 8mil, copper to edge 40mil, drill to drill 8mil, minimum pad ring 10mil, minimum via ring 8mil, stop-mask expansion 4mil, vias tented up to drill 0mil, thermal gap 10mil
Holes 3.2 mm at 2.9,108.05 97.03,108.05 2.9,59.63 97.03,59.63 3.3,3.4 3.3,51.81 72.59,51.85 88.78,51.85 72.59,3.91 88.78,3.91

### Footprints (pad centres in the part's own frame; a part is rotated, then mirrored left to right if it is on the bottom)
RHT03_DHT-22/RA = drill 1.3 pad 1.778 long: DATA -1.27,0; GND 3.81,0; NULL 1.27,0; VDD -3.81,0 | hole 3.25: 0,24.5
BT_MODUL = drill 0.8 long: EN -17.78,-6.985; GND -17.78,-1.905; RX -17.78,3.175; STATE -17.78,5.715; TX -17.78,0.635; VCC -17.78,-4.445
CPOL-RADIAL-2.5MM-5MM = drill 0.7 pad 1.651 square: 1 1.25,0 | drill 0.7 pad 1.651: 2 -1.25,0
0805 = smd 1.016 x 1.422: 1 -0.953,0; 2 0.953,0
C-EL_3,5 = drill 0.813 pad 1.93: C+ 0,0 | drill 0.813 pad 1.93 square: C- 3.493,0
MLW10G = drill 0.914 pad 1.778 square: 1 -5.08,-1.27 | drill 0.914 pad 1.778 octagon: 2 -5.08,1.27; 3 -2.54,-1.27; 4 -2.54,1.27; 5 0,-1.27; 6 0,1.27; 7 2.54,-1.27; 8 2.54,1.27; 9 5.08,-1.27; 10 5.08,1.27
MLW06G = drill 0.914 pad 1.778 square: 1 -2.54,-1.27 | drill 0.914 pad 1.778 octagon: 2 -2.54,1.27; 3 0,-1.27; 4 0,1.27; 5 2.54,-1.27; 6 2.54,1.27
P1206 = smd 0.914 x 1.778: A -1.905,0; K 1.587,0
SO8 = smd 0.6 x 2.2: 1 -1.905,-2.6; 2 -0.635,-2.6; 3 0.635,-2.6; 4 1.905,-2.6; 5 1.905,2.6; 6 0.635,2.6; 7 -0.635,2.6; 8 -1.905,2.6
1206 = smd 1.143 x 1.702: 1 -1.587,0; 2 1.587,0
SO16W = smd 0.6 x 2.2: 1 -4.445,-4.6; 2 -3.175,-4.6; 3 -1.905,-4.6; 4 -0.635,-4.6; 5 0.635,-4.6; 6 1.905,-4.6; 7 3.175,-4.6; 8 4.445,-4.6; 9 4.445,4.6; 10 3.175,4.6; 11 1.905,4.6; 12 0.635,4.6; 13 -0.635,4.6; 14 -1.905,4.6; 15 -3.175,4.6; 16 -4.445,4.6
SO08 = smd 0.66 x 2.032: 1 -1.905,-3.073; 2 -0.635,-3.073; 3 0.635,-3.073; 4 1.905,-3.073; 5 1.905,3.073; 6 0.635,3.073; 7 -0.635,3.073; 8 -1.905,3.073
ATTINY85 = smd 0.6 x 2.286: 1 -1.905,-3.33; 2 -0.635,-3.33; 3 0.635,-3.33; 4 1.905,-3.33; 5 1.905,3.33; 6 0.635,3.33; 7 -0.635,3.33; 8 -1.905,3.33
2X03 = drill 1.016 octagon: 1 -2.54,-1.27; 2 -2.54,1.27; 3 0,-1.27; 4 0,1.27; 5 2.54,-1.27; 6 2.54,1.27
2X02 = drill 1.016 octagon: 1 -1.27,-1.27; 2 -1.27,1.27; 3 1.27,-1.27; 4 1.27,1.27
1X05 = drill 1.016 long: 1 -5.08,0; 2 -2.54,0; 3 0,0; 4 2.54,0; 5 5.08,0
1X03 = drill 1.016 long: 1 -2.54,0; 2 0,0; 3 2.54,0
2X05 = drill 1.016 octagon: 1 -5.08,-1.27; 2 -5.08,1.27; 3 -2.54,-1.27; 4 -2.54,1.27; 5 0,-1.27; 6 0,1.27; 7 2.54,-1.27; 8 2.54,1.27; 9 5.08,-1.27; 10 5.08,1.27
1X01 = drill 1.016 octagon: 1 0,0
ARK500/2 = drill 1.27 pad 3.2 octagon: 1 -2.54,0; 2 2.54,0
ARK500/3 = drill 1.27 pad 3.2 octagon: 1 -5,0; 2 0,0; 3 5,0
LED_3 = drill 0.813 pad 1.778: A -1.27,0 | drill 0.813 pad 1.778 square: K 1.27,0
MOD_APDS9960 = drill 0.9 pad 1.778 offset: P_GND -3.81,-7.62; P_INT 6.35,-7.62; P_SCL 3.81,-7.62; P_SDA 1.27,-7.62; P_VCC -1.27,-7.62; P_VL -6.35,-7.62
MODUL_BMP180 = drill 1.3 pad 1.778 long: GND 1.27,3.81; SCL -1.27,3.81; SDA -3.81,3.81; VCC 3.81,3.81
DS3231 = drill 1.1 pad 2.184 square: 32K 36.83,16.51; SCL1 1.27,14.605 | drill 1.1 pad 2.184: GND1 1.27,6.985; GND2 36.83,3.81; SCL2 36.83,11.43; SDA1 1.27,12.065; SDA2 36.83,8.89; SQW 36.83,13.97; VCC1 1.27,9.525; VCC2 36.83,6.35
64Y = drill 0.813 pad 1.93 octagon: 1 0,2.54; 2 0,-2.54; 3 2.54,0
BIGPIN = drill 1.3 long: P$1 0,0
SOT23-3 = smd 0.8 x 0.9: 1 -0.95,-1; 2 0.95,-1; 3 0,1.1
TO-92 = drill 0.813 octagon: 1 -1.27,0; 2 0,1.905; 3 1.27,0
TO92 = drill 0.813 octagon: 1 1.27,0; 2 0,1.905; 3 -1.27,0
0805' = smd 0.8 x 1.2: 1 -0.9,0; 2 0.9,0
SO08' = smd 0.6 x 2.2: 1 -1.905,-2.6; 2 -0.635,-2.6; 3 0.635,-2.6; 4 1.905,-2.6; 5 1.905,2.6; 6 0.635,2.6; 7 -0.635,2.6; 8 -1.905,2.6
SOT223 = smd 1.219 x 2.235: 1 -2.311,-3.099; 2 0,-3.099; 3 2.311,-3.099 | smd 3.6 x 2.2: 4 0,3.099
KPE242 = drill 0.813 pad 2.184: + -3.81,0 | drill 0.813 pad 2.184 square: - 3.81,0
MICROSD_MODUL = drill 0.8 long: 3,3 -15.24,7.62; CS -15.24,-7.62; GND -15.24,5.08; MISO -15.24,0; MOSI -15.24,-2.54; SCK -15.24,-5.08; VCC -15.24,2.54
SJ_2S-NO = smd 0.635 x 1.27: 1 0,0; 2 0.889,0
EDG-03 = drill 0.813 long: 1 -2.54,-3.81; 2 0,-3.81; 3 2.54,-3.81; 4 2.54,3.81; 5 0,3.81; 6 -2.54,3.81
TSOP = drill 0.8 long: GND -3.81,-9.271; VCC -1.27,-9.271 | drill 0.8 pad 1.27 long: SIGNAL 3.81,-9.271
BLUE_PILL = drill 0.8 long: P$1 -7.62,15.24; P$2 -7.62,12.7; P$3 -7.62,10.16; P$4 -7.62,7.62; P$5 -7.62,5.08; P$6 -7.62,2.54; P$7 -7.62,0; P$8 -7.62,-2.54; P$9 -7.62,-5.08; P$10 -7.62,-7.62; P$11 -7.62,-10.16; P$12 -7.62,-12.7; P$13 -7.62,-15.24; P$14 -7.62,-17.78; P$15 -7.62,-20.32; P$16 -7.62,-22.86; P$17 -7.62,-25.4; P$18 -7.62,-27.94; P$19 -7.62,-30.48; P$20 -7.62,-33.02; P$21 7.62,15.24; P$22 7.62,12.7; P$23 7.62,10.16; P$24 7.62,7.62; P$25 7.62,5.08; P$26 7.62,2.54; P$27 7.62,0; P$28 7.62,-2.54; P$29 7.62,-5.08; P$30 7.62,-7.62; P$31 7.62,-10.16; P$32 7.62,-12.7; P$33 7.62,-15.24; P$34 7.62,-17.78; P$35 7.62,-20.32; P$36 7.62,-22.86; P$37 7.62,-25.4; P$38 7.62,-27.94; P$39 7.62,-30.48; P$40 7.62,-33.02

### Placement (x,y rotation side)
AM2302  31.91,27.15 0 top
BT1  47.94,70.48 0 bottom
C1  94.14,101.92 270 top
C2  69.85,105.25 270 top
C3  90.17,102.23 270 top
C4  94.62,94.14 270 top
C5  90.17,94.61 270 top
C6  24.45,37.31 180 bottom
C7  13.18,41.27 270 bottom
C8  54.61,90.96 180 top
C9  62.71,16.19 180 bottom
C10  56.2,16.19 0 bottom
C11  71.91,37.31 270 bottom
C12  74.61,24.13 0 bottom
C13  72.87,26.67 0 top
C14  88.74,23.65 0 top
C15  41.59,24.45 0 bottom
C16  41.59,17.3 270 top
C17  67.63,41.27 180 top
C18  41.59,40.8 180 top
C19  67.63,34.61 0 bottom
C20  67.63,27.62 90 top
C21  49.37,55.72 90 bottom
C22  41.59,48.58 0 bottom
C23  67.63,17.3 0 bottom
C24  24.61,55.72 90 bottom
C25  60.01,55.72 90 top
C26  76.84,55.72 90 top
C27  82.39,55.72 0 bottom
C28  19.21,55.72 0 top
CON1  94.14,73.18 90 top
CON2  12.07,16.83 90 bottom
CON3  10.79,98.11 90 top
D1  78.26,46.51 180 top
D2  78.26,44.13 180 top
EEPROM  62.87,104.46 90 top
FUSE  15.4,65.41 0 bottom
IC1  31.91,41.75 180 bottom
IC2  55.25,25.72 270 bottom
IC3  80.17,27.15 180 bottom
IC4  87,28.58 0 bottom
ISP  86.36,38.89 90 top
JP1  59.37,82.55 90 bottom
JP2  42.86,84.93 90 bottom
JP3  80.01,38.89 270 top
JP4  55.25,41.59 270 top
JP5  41.59,97.95 270 bottom
JP6  76.84,38.89 270 top
JP7  54.29,79.53 90 top
JP8  54.29,82.07 90 top
JP9  54.29,84.61 90 top
JP10  15.4,3.97 0 bottom
JP17  38.26,80.49 0 top
JP20  40.32,108.43 90 top
K1  48.58,7.14 270 bottom
K3  85.41,17.3 0 top
K4  75.25,17.3 0 top
K5  48.58,17.3 270 bottom
KON-DS18B20  5.08,82.55 90 bottom
KON-PWR  5.08,67.94 90 bottom
LED1  20.48,7.62 0 top
LED2  20.48,24.29 0 top
LED3  20.48,16.03 0 top
LED4  13.97,32.07 180 top
MOD1  31.91,11.27 0 top
MOD2  80.96,82.07 0 top
MOD3  91.12,109.22 270 bottom
P1  60.01,91.92 270 bottom
PIN1  56.36,3.02 0 top
PIN2  42.7,59.37 0 top
Q1  18.89,12.06 90 top
Q2  18.41,20 90 top
Q3  65.41,82.07 270 top
Q4  65.25,96.68 180 top
R1  22.54,46.51 0 bottom
R2  22.54,43.97 0 bottom
R3  24.29,41.43 0 bottom
R4  10.79,29.69 90 bottom
R5  13.97,85.57 270 top
R6  29.37,23.81 0 bottom
R7  66.36,86.36 0 top
R8  10k  [0805']  22.38,12.06 90 top
R9  10k  [0805']  16.67,29.05 270 bottom
R10  10k  [0805']  21.59,19.69 90 top
R11  10k  [0805']  19.37,27.78 270 bottom
R12  49.69,39.05 0 bottom
R13  49.69,36.51 0 bottom
R14  49.69,41.59 0 bottom
R15  47.62,31.91 180 bottom
R16  48.26,24.92 90 bottom
R17  46.67,28.42 270 bottom
R18  72.39,34.45 0 bottom
R19  72.39,32.38 0 bottom
R20  72.39,30.16 0 bottom
R21  79.22,20.32 0 bottom
R22  83.98,25.72 180 top
R23  74.3,37.31 270 bottom
R24  83.34,23.5 180 top
R25  84.14,46.51 0 top
R26  84.14,44.13 180 top
RAM1  47C16  [SO08']  83.66,101.28 90 top
RAM2  47C16  [SO08']  83.66,94.3 90 top
REFUSE-PB3  76.2,32.38 0 top
REG1  61.59,7.3 180 bottom
REP1  23.81,64.45 0 top
SD1  19.68,89.06 90 bottom
SJ-SCL1  83.34,41.59 0 bottom
SW1  31.91,13.02 0 bottom
TSOP1  14.45,46.67 0 top
U$1  42.55,75.72 180 top

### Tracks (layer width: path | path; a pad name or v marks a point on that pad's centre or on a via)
0V  (via drill 0.7)
  Top 0.61: 90.17,96.2 C5.1 | 94.62,95.41 C4.2 | C2.1 65.47,106.2 EEPROM.4 62.87,106.36 62.87,103.82 EEPROM.7 | 52.07,66.83 48.26,66.83
  Top 0.813: C3.1 RAM1.4 86.26,105.73 73.03,105.73 73.03,106.2 C2.1 | RAM2.4 94.62,96.2 | RAM2.4 90.17,96.2 | RAM2.4 RAM2.3
  Top 1.016: BT1.GND 62.39,68.58 62.39,66.83 52.07,66.83
  Top 1.27: 94.62,96.2 C4.2 | C3.1 96.52,103.19 96.52,103.17 | 96.52,103.17 96.52,95.41 94.62,95.41 | KON-PWR.2 KON-DS18B20.1 | JP2.1 42.86,66.83 | 42.86,66.83 42.86,63.02 U$1.P$22 | 48.26,66.83 42.86,66.83 | P1.2 67.47,91.92 67.47,96.68 Q4.3 | v71.28,90.33 82.23,90.33 MOD2.GND | C1.2 96.52,103.17
  Bottom 0.61: JP5.7 44.77,95.41 44.77,91.44 40.16,91.44 40.16,79.85 JP2.1 | C24.2 24.61,63.02 24.77,63.02
  Bottom 1.016: KON-DS18B20.1 9.53,77.55 CON3.2
  Bottom 1.27: KON-PWR.2 24.77,70.48 | 24.77,70.48 SD1.GND | U$1.P$22 31.43,63.02 31.43,60.64 24.77,60.64 24.77,63.02 24.77,70.48 | 87,65.56 87,72.07 MOD3.GND2 89.22,74.29 89.22,79.37 82.23,79.37 MOD2.GND 82.23,95.39 C4.2 | 87,65.56 95.41,65.56 CON1.1 | 87,65.56 70.17,65.56 67.15,68.58 BT1.GND | Q4.3 71.28,96.68 v71.28,90.33
+3V  (via drill 0.7)
  Top 0.61: v69.69,70.01 69.69,75.72 v82.55,75.72 | v87.31,75.72 CON1.8
  Bottom 0.61: U$1.P$23 46.04,65.56 46.04,66.83 62.39,66.83 62.39,69.85 69.69,69.85 v69.69,70.01 | v82.55,75.72 v87.31,75.72
+5V  (via drill 0.7)
  Top 0.61: 88.9,101.92 88.9,101.44 | 90.17,101.44 C3.2 | RAM2.2 C5.2 | RAM1.2 83.66,100.65 | EEPROM.3 EEPROM.2 EEPROM.1 | EEPROM.1 EEPROM.8 | EEPROM.1 60.17,102.55 v60.17,98.9 | 37.15,107.47 32.39,107.47 | 85.25,85.88 MOD2.VCC
  Top 0.813: 88.9,101.92 RAM1.3 86.26,100.81 | 88.9,101.44 90.17,101.44 | RAM1.2 86.26,100.81 | RAM1.8 83.66,99.38 | 83.66,99.38 83.66,100.65 83.66,104.3 C2.2 65.47,104.3 EEPROM.1 | 83.66,100.81 86.26,100.81 | 83.66,99.38 83.66,93.66 | 83.66,93.66 RAM2.2 | RAM2.8 83.66,92.39 | 83.66,92.39 83.66,93.66 | 84.77,90.49 83.66,90.49 83.66,92.39
  Top 1.27: Q3.1 R7.1 65.41,88.74 69.53,88.74 69.53,98.9 | v60.17,98.9 69.53,98.9 | 22.23,107.47 9.53,107.47 CON3.6 | 37.15,107.47 38.42,107.47 38.42,106.36 v45.88,106.36 47.78,106.36 47.78,103.66 U$1.P$18 | 32.39,107.47 22.23,107.47 | MOD2.VCC 84.77,90.49 | v22.23,92.87 22.23,107.47 | MOD3.VCC2 85.25,72.39 85.25,85.88 | SD1.VCC 22.23,67.79 20,67.79 REP1.+ | 69.53,98.9 69.53,103.98
  Bottom 0.61: JP2.5 45.88,90.01 45.88,97.95 | 45.88,97.95 v45.88,106.36 | MOD2.VCC 84.77,85.72 | JP5.5 45.88,97.95
  Bottom 1.27: v60.17,98.9 56.36,98.9 56.36,103.66 U$1.P$18 | 84.77,85.72 92.87,85.72 CON1.10 | SD1.VCC v22.23,92.87 | FUSE.1 16.99,64.45 REP1.+
+PWR
  Bottom 1.27: KON-PWR.1 FUSE.2
B2_0V  (via drill 0.7)
  Top 0.61: SW1.3 28.1,9.21 MOD1.P_GND | v20.96,37.46 20.96,39.53 18.26,39.53 v18.26,48.58 C28.1
  Bottom 0.61: SW1.3 SW1.2 SW1.1 39.05,9.21 39.05,24.45 | CON2.1 10.8,1.9 28.1,1.9 MOD1.P_GND | IC1.8 36.35,48.58 | 36.35,48.58 30,48.58 | IC1.3 30,48.58 | IC1.2 28.73,48.58 | 28.73,48.58 30,48.58 | IC1.1 27.46,48.58 | 27.46,48.58 28.73,48.58 | TSOP1.GND 10.64,42.07 | 10.64,42.07 10.64,48.58 v18.26,48.58 24.61,48.58 | 24.61,48.58 27.46,48.58 | AM2302.GND 39.05,27.15 | 39.05,27.15 39.05,48.58 | 39.05,48.58 36.35,48.58 | 39.05,24.45 39.05,27.15 | C7.1 13.18,42.07 10.64,42.07 | C6.1 23.5,37.46 v20.96,37.46 | 39.05,48.58 C22.2 | C15.2 39.05,24.45 | C24.1 24.61,48.58
B2_+3V  (via drill 0.7)
  Top 0.61: R10.1 21.59,19.05 Q2.1 19.42,16.03 LED3.A | R8.1 22.38,11.11 Q1.1 v25.4,11.11
  Bottom 0.61: MOD1.P_VCC 30.64,7.14 25.56,7.14 | 25.56,7.14 MOD1.P_VL 19.21,3.65 LED1.A LED3.A 19.21,21.27 | LED4.A 27.46,32.07 IC1.16 27.46,37.31 C6.2 | 15.4,32.07 LED4.A | 15.24,21.27 15.24,20.48 14.13,19.37 CON2.8 | 15.24,21.27 19.21,21.27 | LED4.A 15.24,21.27 | v25.4,11.11 25.56,11.11 25.56,7.14 | 19.21,21.27 LED2.A
B2_+5V  (via drill 0.7)
  Top 0.61: CON2.10 13.34,28.73 v21.11,28.73 21.11,34.13 13.18,34.13 TSOP1.VCC
  Bottom 0.61: R6.2 28.42,27.15 AM2302.VDD 28.1,28.73 v21.11,28.73 | C7.2 TSOP1.VCC | 21.11,28.63 v21.11,28.73 | R9.1 18.1,29.95 18.1,28.73 19.37,28.73 R11.1 21.11,28.68 v21.11,28.73
B2_INFRA
  Bottom 0.61: CON2.5 8.89,16.83 8.89,33.81 18.26,33.81 TSOP1.SIGNAL
B2_INT_POHYB  (via drill 0.7)
  Top 0.61: v8.89,1.9 38.26,1.9 MOD1.P_INT
  Bottom 0.61: CON2.3 8.89,14.29 v8.89,1.9
B2_LED-BK
  Bottom 0.61: IC1.4 31.27,44.45 26.51,44.45 24.45,46.51 R1.1
B2_LED-GK
  Bottom 0.61: IC1.6 33.81,41.91 25.24,41.91 R3.1
B2_LED-RK
  Bottom 0.61: IC1.5 32.54,43.18 25.4,43.18 24.61,43.97 R2.1
B2_LED_I
  Bottom 0.61: CON2.9 R4.1
B2_NC3
  Bottom 0.61: CON2.6 14.61,16.83 15.4,16.03 JP10.1
B2_SCL_H  (via drill 0.7)
  Top 0.61: 17.46,20 17.47,20 17.47,17.14 14.62,14.29 CON2.4 | 17.46,20 Q2.3 | 17.46,20 17.46,26.83 v21.43,26.83
  Bottom 0.61: v21.43,26.83 19.37,26.83 R11.2
B2_SCL_L  (via drill 0.7)
  Top 0.61: MOD1.P_SCL 35.72,14.29 37.62,14.29 | 37.62,14.29 39.21,14.29 | 39.21,14.29 39.21,40.8 | 39.21,40.8 v35.88,40.8 | Q2.2 21.59,20.95 R10.2 23.34,20.58 23.34,19.05 v25.56,19.05 | 37.62,14.29 v37.62,13.33 | C18.2 39.21,40.8 | C16.2 41.59,14.29 39.21,14.29
  Bottom 0.61: v35.88,40.8 30,40.8 IC1.14 | v37.62,13.33 37.62,19.05 v25.56,19.05
B2_SDA_H  (via drill 0.7)
  Top 0.61: CON2.2 17.62,11.75 | 17.62,11.75 17.79,11.75 Q1.3 | v16.35,23.18 15.72,23.18 15.72,19.05 v16.03,18.73 | v17.62,14.45 17.62,11.75
  Bottom 0.61: 16.35,28.2 16.35,28.15 | 16.35,28.15 v16.35,23.18 | R9.2 16.35,28.15 | v16.03,18.73 17.62,17.14 v17.62,14.45
B2_SDA_L  (via drill 0.7)
  Top 0.61: MOD1.P_SDA 33.18,11.59 26.67,11.59 | v7.78,35.08 7.14,35.08 7.14,9.68 26.67,9.68 26.67,11.59 | Q1.2 22.38,13.01 R8.2 26.67,12.96 26.67,11.59
  Bottom 0.61: IC1.15 28.73,39.53 15.4,39.53 15.4,35.08 v7.78,35.08
B2_VLHKOMER  (via drill 0.7)
  Top 0.61: CON2.7 8.89,19.37 8.89,30.48 v19.37,30.48
  Bottom 0.61: R6.1 30.32,27.15 AM2302.DATA 30.64,30.48 v19.37,30.48
B3_+3V  (via drill 0.7)
  Top 0.61: C18.1 42.55,34.29 v48.74,34.29
  Top 0.813: v48.74,27.94 v48.74,34.29 | v54.77,26.83 54.95,26.83 C10.1
  Bottom 0.61: R14.2 48.74,48.58 | 48.74,48.58 C22.1 | C21.1 49.37,48.58 48.74,48.58
  Bottom 0.813: 54.93,16.19 C10.1 | R14.2 R12.2 R13.2 v48.74,34.29 | v48.74,27.94 48.74,27.62 IC2.8 54.77,27.62 v54.77,26.83
  Bottom 1.27: 54.93,16.19 54.93,18.26 59.37,18.26 59.37,13.49 61.6,13.49 REG1.2
B3_+5V  (via drill 0.7)
  Top 0.61: K5.1 41.59,19.84 C16.1 | 62.55,41.59 62.55,41.27 C17.2 | C25.1 60.01,41.59
  Top 0.813: 62.55,31.11 v51.28,31.11 51.28,19.84 K5.1 | 62.55,31.11 62.55,41.59 60.01,41.59 JP4.6 | C20.2 67.63,31.11 62.55,31.11
  Bottom 0.813: R15.2 48.58,31.11 v51.28,31.11
  Bottom 1.27: K5.1 63.98,19.84 63.98,16.19 C9.1 | REG1.3 63.96,10.4 C9.1 | C23.2 63.96,17.3 C9.1
B3_GND  (via drill 0.7)
  Top 0.813: C9.2 61.28,16.19
  Top 1.27: C10.2 C9.2 | 61.28,16.19 v61.28,21.59
  Bottom 0.61: C19.2 62.55,34.61
  Bottom 0.813: JP4.8 62.55,39.05 62.55,34.61 62.55,21.59 v61.28,21.59 52.17,21.59 IC2.5 48.26,23.81 R16.1
  Bottom 1.27: 57.45,10.4 52.86,10.4 52.86,4.6 K1.2 | REG1.1 57.45,10.4 | 57.45,10.4 C10.2
B3_KOM_A
  Bottom 0.61: C15.1 44.77,24.45
  Bottom 0.813: R15.1 R17.1 | IC2.6 56.36,25.08 56.36,29.37 R17.1 | R17.1 44.77,29.37 44.77,24.45 44.77,9.68 K1.1
B3_KOM_B
  Bottom 0.813: IC2.7 48.26,26.35 R16.2 46.2,25.88 | R17.2 46.2,27.46 46.2,25.88 | 46.2,25.88 46.2,14.76 K5.2
B3_RS485-RX
  Bottom 0.813: R13.1 JP4.9 53.98,33.02 59.85,33.02 59.85,27.62 IC2.1
B3_RS485-SMER  (via drill 0.7)
  Top 0.61: JP4.5 55.25,40.32 57.94,40.32
  Top 0.813: 57.94,40.32 61.12,40.32 v61.12,34.13
  Bottom 0.813: R14.1 JP4.5 | v61.12,34.13 61.12,25.08 IC2.3 IC2.2
B3_RS485-TX  (via drill 0.7)
  Top 0.813: v60.48,23.49 57.79,23.49 v57.79,29.53 | v52.55,33.81 52.39,33.81 52.39,39.05 JP4.7
  Bottom 0.813: JP4.7 R12.1 | IC2.4 60.48,23.81 v60.48,23.49 | v57.79,29.53 57.79,31.27 52.55,31.27 v52.55,33.81
B4_+5V  (via drill 0.7)
  Top 0.813: JP3.3 ISP.2 | C14.2 90.81,23.65 90.81,20.32 | 90.81,20.32 90.81,14.92 72.71,14.92 K4.1 | v89.69,20.32 90.81,20.32 | C20.1 C13.C+
  Bottom 0.61: C19.1 68.58,34.45 R18.2 | C23.1 K4.1
  Bottom 0.813: JP3.3 JP6.3 R23.2 C11.2 71.44,36.35 R18.2 R19.2 R20.2 71.44,26.67 C13.C+ 72.87,24.13 | 72.87,24.13 C12.2 | 72.87,24.13 72.87,21.75 | 72.87,21.75 72.87,17.3 K4.1 | IC3.8 R21.2 78.26,21.75 72.87,21.75 | IC4.8 90.81,31.9 90.81,20.32 v89.69,20.32
B4_A
  Top 0.813: R24.1 84.3,17.3 K3.1
  Bottom 0.813: IC3.6 80.8,20.32 | 80.8,20.32 R21.1 | 80.8,20.32 82.87,20.32 K3.1
B4_B  (via drill 0.7)
  Top 0.813: v79.53,22.22 79.53,17.3 K4.2 | R22.2 79.53,25.72 v79.53,22.22 | R24.2 79.53,23.49 v79.53,22.22
  Bottom 0.813: IC3.7 v79.53,22.22
B4_GND
  Top 0.61: 76.68,41.43 D2.K D1.K 76.68,54.77 C26.1 | C17.1 68.58,41.43 JP6.1
  Top 0.813: ISP.6 JP3.1 JP6.1 76.68,41.43 74.61,41.43 74.61,26.67 C13.C- | K3.2 87.79,17.3 C14.1 87.79,25.72 R22.1
  Bottom 0.813: C11.1 71.91,41.43 JP6.1 | C13.C- 76.36,26.03 | 76.36,26.03 76.36,24.13 C12.1 | 76.36,26.03 82.07,26.03 IC3.5 85.09,24.07 | IC4.4 85.09,24.07 | 85.09,24.07 85.09,20.48 87.95,20.48 K3.2
BLUE-RX
  Top 0.61: JP1.2 60.64,73.66 BT1.RX
BLUE-TX
  Bottom 0.61: JP1.4 62.39,83.82 62.39,71.12 BT1.TX
BT-ON
  Top 0.61: R7.2 Q3.2
  Bottom 0.61: Q3.2 67.31,87.15 47.94,87.15 47.94,71.6 38.89,71.6 38.89,75.72 U$1.P$27
BT-PWR
  Top 0.61: Q3.3 65.56,80.8
  Top 1.27: 65.56,80.8 65.56,79.37 68.1,79.37 68.1,66.04 BT1.VCC
BZUK
  Top 0.61: C8.2 U$1.P$13
BZUK-C
  Top 0.61: C8.1 55.56,91.92 P1.1
BZUK-DRAIN  (via drill 0.7)
  Top 0.61: v26.04,76.83 26.04,64.45 REP1.- 27.62,55.72 C28.2 | v26.04,87.15 40.32,87.15 40.32,86.2 45.4,86.2 45.4,87.15 56.36,87.15 56.36,88.26 59.85,91.76 59.85,94.77 Q4.2
  Bottom 0.61: v26.04,76.83 v26.04,87.15
BZUK-GATE
  Bottom 0.813: P1.3 60.01,94.77 62.07,94.77 Q4.1
DIS-RX
  Bottom 0.61: CON3.1 29.69,95.57 29.69,70.64 U$1.P$25
DIS-TX
  Bottom 0.61: CON3.5 31.43,100.65 31.43,73.18 U$1.P$26
DS18B20  (via drill 0.7)
  Top 0.61: KON-DS18B20.2 13.97,82.55 | 13.97,82.55 R5.2 | v39.53,70.33 39.53,74.45 30,74.45 30,78.58 13.97,78.58 13.97,82.55
  Bottom 0.61: U$1.P$5 50.17,70.33 v39.53,70.33
DS18B20-PWR
  Top 0.61: KON-DS18B20.3 13.97,87.55 | 13.97,87.55 R5.1 | U$1.P$16 50.17,98.27 46.2,98.27 46.2,104.46 37.62,104.46 37.62,89.69 13.97,89.69 13.97,87.55
I2C-SCL  (via drill 0.7)
  Top 0.61: RAM2.6 v77.63,94.93 78.11,94.93 | RAM1.6 v77.63,101.92 | 56.36,100.65 56.36,93.5 U$1.P$14 46.2,93.5 46.2,92.87 JP5.9 | 56.36,100.65 56.36,105.09 EEPROM.6 | v57.94,100.65 56.36,100.65 | CON1.4 92.87,70.48 79.69,70.48 MOD3.SCL2
  Bottom 0.61: v77.63,101.92 77.63,100.65 | 77.63,100.65 v57.94,100.65 | MOD3.SCL2 MOD2.SCL 79.69,94.93 v77.63,94.93 77.63,100.65
I2C-SDA  (via drill 0.7)
  Top 0.61: RAM1.5 74.45,103.19 v74.45,102.55 v74.45,96.2 RAM2.5 | EEPROM.5 57.94,106.36 | 57.94,106.36 54.93,106.36 54.93,96.2 50.17,96.2 U$1.P$15 44.93,96.04 44.93,100.49 JP5.3 | CON1.2 92.87,67.47 v82.23,67.47 | v57.94,107.95 57.94,106.36
  Bottom 0.61: v74.45,96.2 74.45,85.88 MOD2.SDA 77.15,77.31 72.71,77.31 72.71,67.47 v82.23,67.47 MOD3.SDA2 | v74.45,102.55 57.94,102.55 v57.94,107.95
INFRA  (via drill 0.7)
  Top 0.61: v72.71,82.39 v83.66,82.39
  Bottom 0.305: 94.14,74.45 91.6,74.45
  Bottom 0.61: U$1.P$17 54.93,101.12 54.93,97.47 61.75,97.47 61.75,98.58 72.71,98.58 v72.71,82.39 | v83.66,82.39 90.49,82.39 90.49,74.45 91.6,74.45 | CON1.5 94.14,74.45
INT_POHYB
  Bottom 0.61: U$1.P$1 81.44,60.48 | 81.44,60.48 88.9,60.48 88.9,63.82 97.79,63.82 97.79,70.64 CON1.3 | C27.2 81.44,60.48
  Bottom 0.813: U$1.P$1 50.17,56.67 C21.2
INT_RTC  (via drill 0.7)
  Top 0.61: v77.15,61.75 MOD3.SQW
  Bottom 0.61: U$1.P$2 63.5,63.02 63.5,61.75 v77.15,61.75
KOM-RX
  Top 0.61: JP1.3 56.52,83.82 56.52,75.72 U$1.P$7 47.15,75.72 47.15,84.93 JP2.3
KOM-TX
  Top 0.61: JP1.1 58.1,73.18 U$1.P$6 50.17,73.02 45.4,73.02 45.4,82.39 JP2.2
LED_I
  Top 0.61: CON1.9 97.63,78.26 97.63,63.82 88.9,63.82 88.9,60.48 76.84,60.48 | 76.84,60.48 60.01,60.48 | 60.01,60.48 53.82,60.48 53.82,65.56 U$1.P$3 | C25.2 60.01,60.48 | C26.2 76.84,60.48
MISO  (via drill 0.7)
  Top 0.61: U$1.P$30 v19.69,83.34
  Bottom 0.61: v19.69,83.34 SD1.MISO
MOSI  (via drill 0.7)
  Top 0.61: U$1.P$29 v17.15,80.8
  Bottom 0.61: v17.15,80.8 SD1.MOSI
MOSI-ISP
  Top 0.406: 86.36,42.39 86.36,40.64
  Top 0.61: R26.1 86.36,44.13 86.36,42.39 | 86.36,40.64 86.36,40.16 ISP.4
  Bottom 0.813: IC4.5 83.5,31.9 83.5,38.26 84.14,38.89 ISP.4
N$1  (via drill 0.7)
  Top 0.61: v15.56,46.51 5.56,46.51 5.56,7.3 16.67,7.3 18.57,5.4 21.75,5.4 LED1.K
  Bottom 0.61: 21.59,46.67 R1.2 v15.56,46.51
N$2  (via drill 0.7)
  Top 0.61: v15.56,44.45 15.56,35.24 22.54,35.24 22.54,24.29 LED2.K
  Bottom 0.61: R2.2 21.11,44.45 v15.56,44.45
N$3  (via drill 0.7)
  Top 0.61: v21.11,41.59 23.65,41.59 23.65,21.75 27.15,21.75 27.15,16.03 LED3.K
  Bottom 0.61: R3.2 21.11,41.43 v21.11,41.59
N$4
  Bottom 0.305: 5.87,103.66 30.64,103.66 30.64,110.01 5.87,110.01 5.87,103.66
N$5
  Bottom 0.61: R4.2 10.8,32.07 LED4.K
N$6
  Top 0.61: D2.A R26.2 | R26.2
N$7  (via drill 0.7)
  Top 0.61: v29.05,33.97 24.92,33.97 24.92,23.02 29.37,23.02 SW1.4
  Bottom 0.61: IC1.11 33.81,33.97 v29.05,33.97
N$8
  Top 0.813: RAM2.1 94.62,92.39 C4.1
N$9  (via drill 0.7)
  Top 0.61: v32.54,31.91 26.19,31.91 26.19,24.13 31.91,24.13 SW1.5
  Bottom 0.61: IC1.10 35.08,31.91 v32.54,31.91
N$10  (via drill 0.7)
  Top 0.61: v36.83,32.7 37.78,32.7 37.78,16.83 SW1.6
  Bottom 0.61: IC1.9 36.35,32.7 v36.83,32.7
N$12
  Top 0.813: JP6.2 JP3.2
  Bottom 0.61: SJ-SCL1.2 82.46,39.59 81.76,38.89 JP3.2
  Bottom 0.813: R23.1 74.3,38.89 JP6.2
N$13
  Top 0.61: D1.A R25.1 | R25.1
N$17
  Top 0.813: RAM1.1 94.14,99.38 C1.1
NC1
  Bottom 0.61: U$1.P$8 51.59,78.26 52.86,79.53 JP7.1
NC2
  Bottom 0.61: U$1.P$9 51.59,80.8 52.86,82.07 JP8.1
NC3  (via drill 0.7)
  Top 0.61: v71.28,72.23 71.28,69.06 v75.41,69.06 | v88.74,69.06 v78.58,69.06
  Bottom 0.61: v71.28,72.23 71.28,78.26 63.82,78.26 63.82,85.88 54.29,85.88 JP9.1 53.02,84.61 51.75,83.34 U$1.P$10 | CON1.6 91.44,73.18 90.65,72.39 90.65,69.06 v88.74,69.06 | v78.58,69.06 v75.41,69.06
NC4  (via drill 0.7)
  Top 0.61: v47.78,108.27 v43.97,108.27
  Bottom 0.61: U$1.P$12 47.78,88.42 v47.78,108.27 | v43.97,108.27 43.97,103.03 JP5.1
NC5
  Bottom 0.61: U$1.P$28 36.04,78.26 JP17.1
NC6
  Bottom 0.61: U$1.P$36 36.35,98.58 38.26,100.49 JP5.4
RS485-RX
  Bottom 0.61: U$1.P$33 36.35,90.96 38.26,92.87 JP5.10
RS485-SMER
  Bottom 0.61: U$1.P$35 36.35,96.04 38.26,97.95 JP5.6
RS485-TX
  Bottom 0.61: U$1.P$34 36.35,93.5 38.26,95.41 JP5.8
RST-ISP  (via drill 0.7)
  Top 0.813: ISP.5 90.81,41.43 90.81,29.53 v88.74,29.53
  Bottom 0.813: v88.74,29.53 88.9,29.53 IC4.1
SCK  (via drill 0.7)
  Top 0.61: v17.15,85.88 U$1.P$31
  Bottom 0.61: SD1.SCK 14.61,85.88 v17.15,85.88
SCK-ISP  (via drill 0.7)
  Top 0.61: R25.2 89.22,46.51 v89.22,44.93
  Top 0.813: ISP.3 89.54,38.89 89.54,32.23 86.04,32.23 | 86.04,32.23 v86.04,29.53 | v80.65,32.23 86.04,32.23
  Bottom 0.61: v86.04,29.53 87.63,29.53 IC4.7 | v89.22,44.93 89.22,38.89 ISP.3
  Bottom 0.813: IC3.2 80.17,30.22 | 80.17,30.22 IC3.3 80.65,30.22 v80.65,32.23 | R20.1 73.34,28.42 80.17,28.42 80.17,30.22
SD_CS  (via drill 0.7)
  Top 0.61: v19.84,88.42 U$1.P$32
  Bottom 0.61: SD1.CS 12.07,88.42 v19.84,88.42
SPOJKA
  Bottom 0.61: JP5.2 JP20.1
TINY-PB4
  Bottom 0.813: R18.1 82.07,34.45 IC3.4 82.07,27.94 86.36,27.94 IC4.3
TL1  (via drill 0.7)
  Top 0.813: v87.63,28.1 78.26,28.1 v78.26,32.23
  Bottom 0.813: IC4.2 v87.63,28.1 | v78.26,32.23 78.26,32.38 REFUSE-PB3.1 R19.1
  Bottom 1.016: v78.26,32.23 IC3.1
VCC2-MISO-ISP
  Bottom 0.61: SJ-SCL1.1 83.34,46.51 | 83.34,46.51 90.81,46.51 | C27.1 83.34,46.51
  Bottom 0.813: 90.81,46.51 90.81,36.35 ISP.1 87.47,36.35 87.47,33.97 86.36,33.97 IC4.6
VLHKOMER  (via drill 0.7)
  Top 0.61: U$1.P$11 63.02,85.88 v63.02,89.06 | v70.33,80.17 70.33,77.63 v82.55,77.63 | v87.31,77.63 87.31,77.47 90.01,77.47 90.01,84.3 v97.31,84.3
  Bottom 0.61: v63.02,89.06 63.02,88.74 70.33,88.74 v70.33,80.17 | v82.55,77.63 v87.31,77.63 | v97.31,84.3 97.31,75.72 CON1.7

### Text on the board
Bottom: Astrohodiny / s meteostanici | ver.7
tPlace: EEPROM | Displej | EERAM | N | PWR | DATA | P | TLAK | GND | +5V | BUZZ | http://meteo.AstroMiK.org | 1 | Tx | Vlhkost | Rx | G | D | V | 1 | V | B | V | B | A | G | A | RS485 | G
bPlace: RTC | 1 | 5V | 3V | Tx | Rx | G | Micro SD | Bluetooth | GND | +5V | 1 | C | B | A | V | B | V | B | A | G | A | G
nuzky: ✂ | ✂ | ✂
T_nam_docu: G | S | D | K | A | A | A | A | K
